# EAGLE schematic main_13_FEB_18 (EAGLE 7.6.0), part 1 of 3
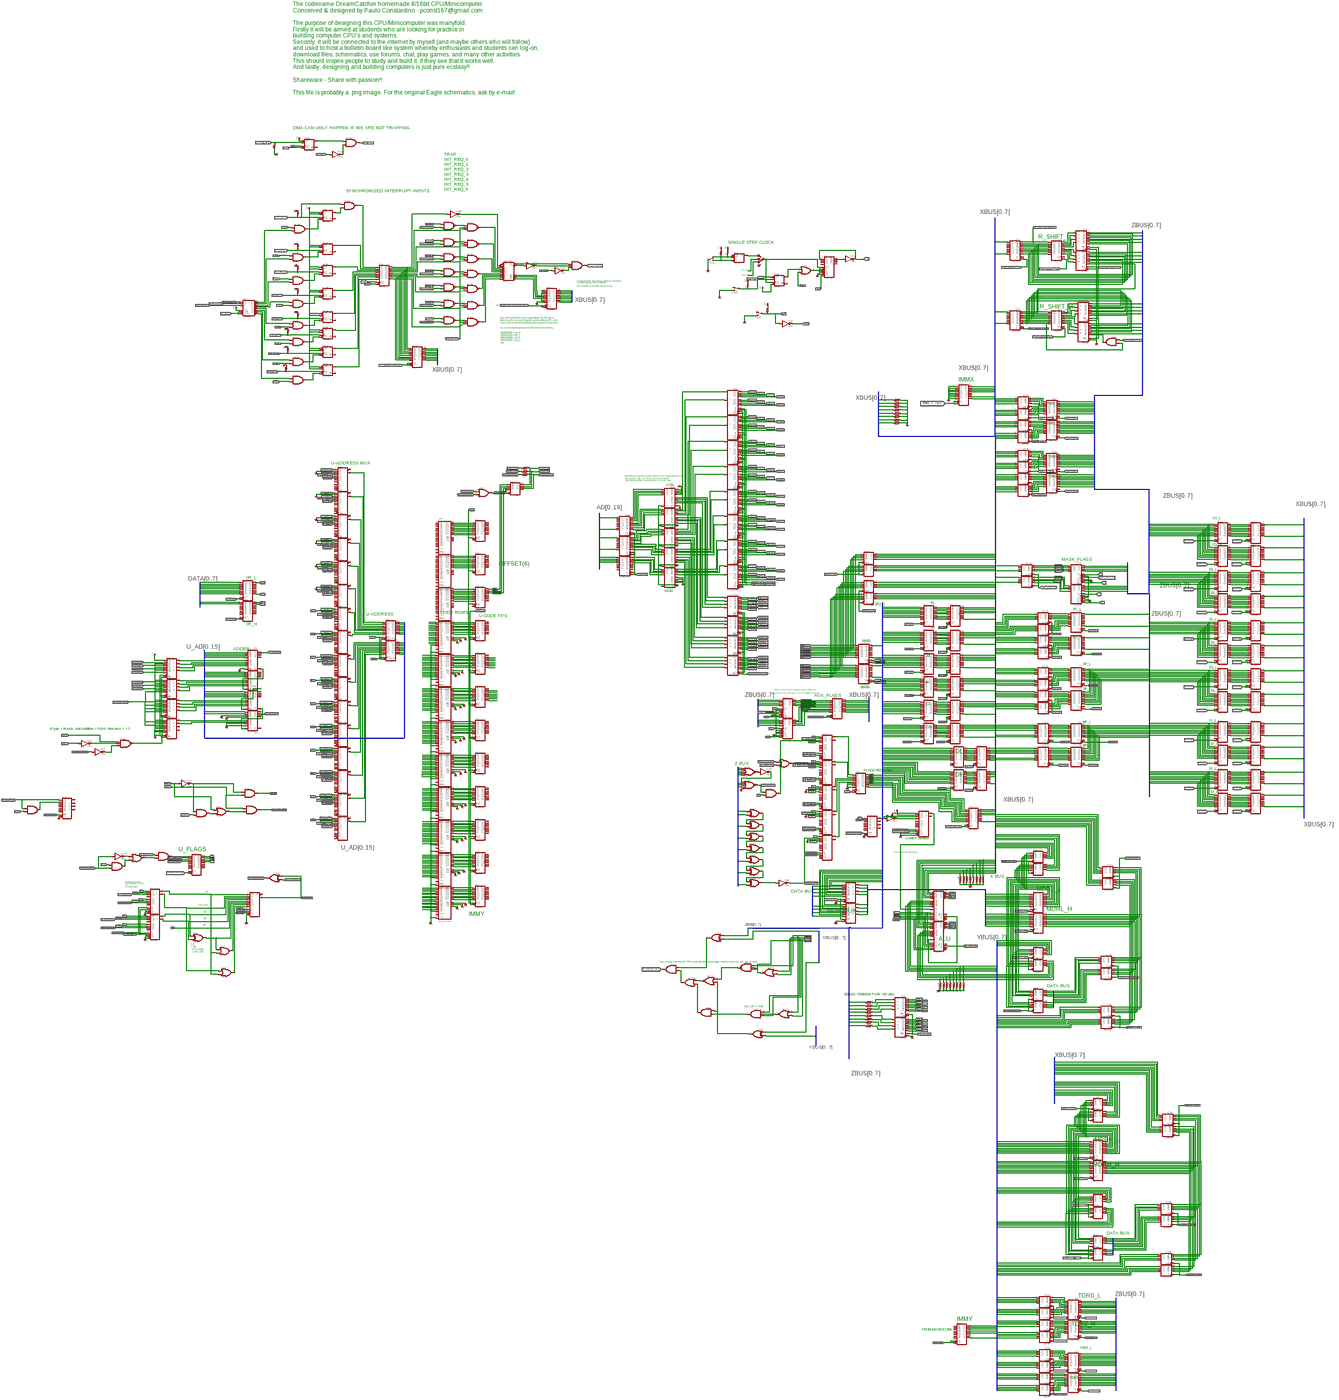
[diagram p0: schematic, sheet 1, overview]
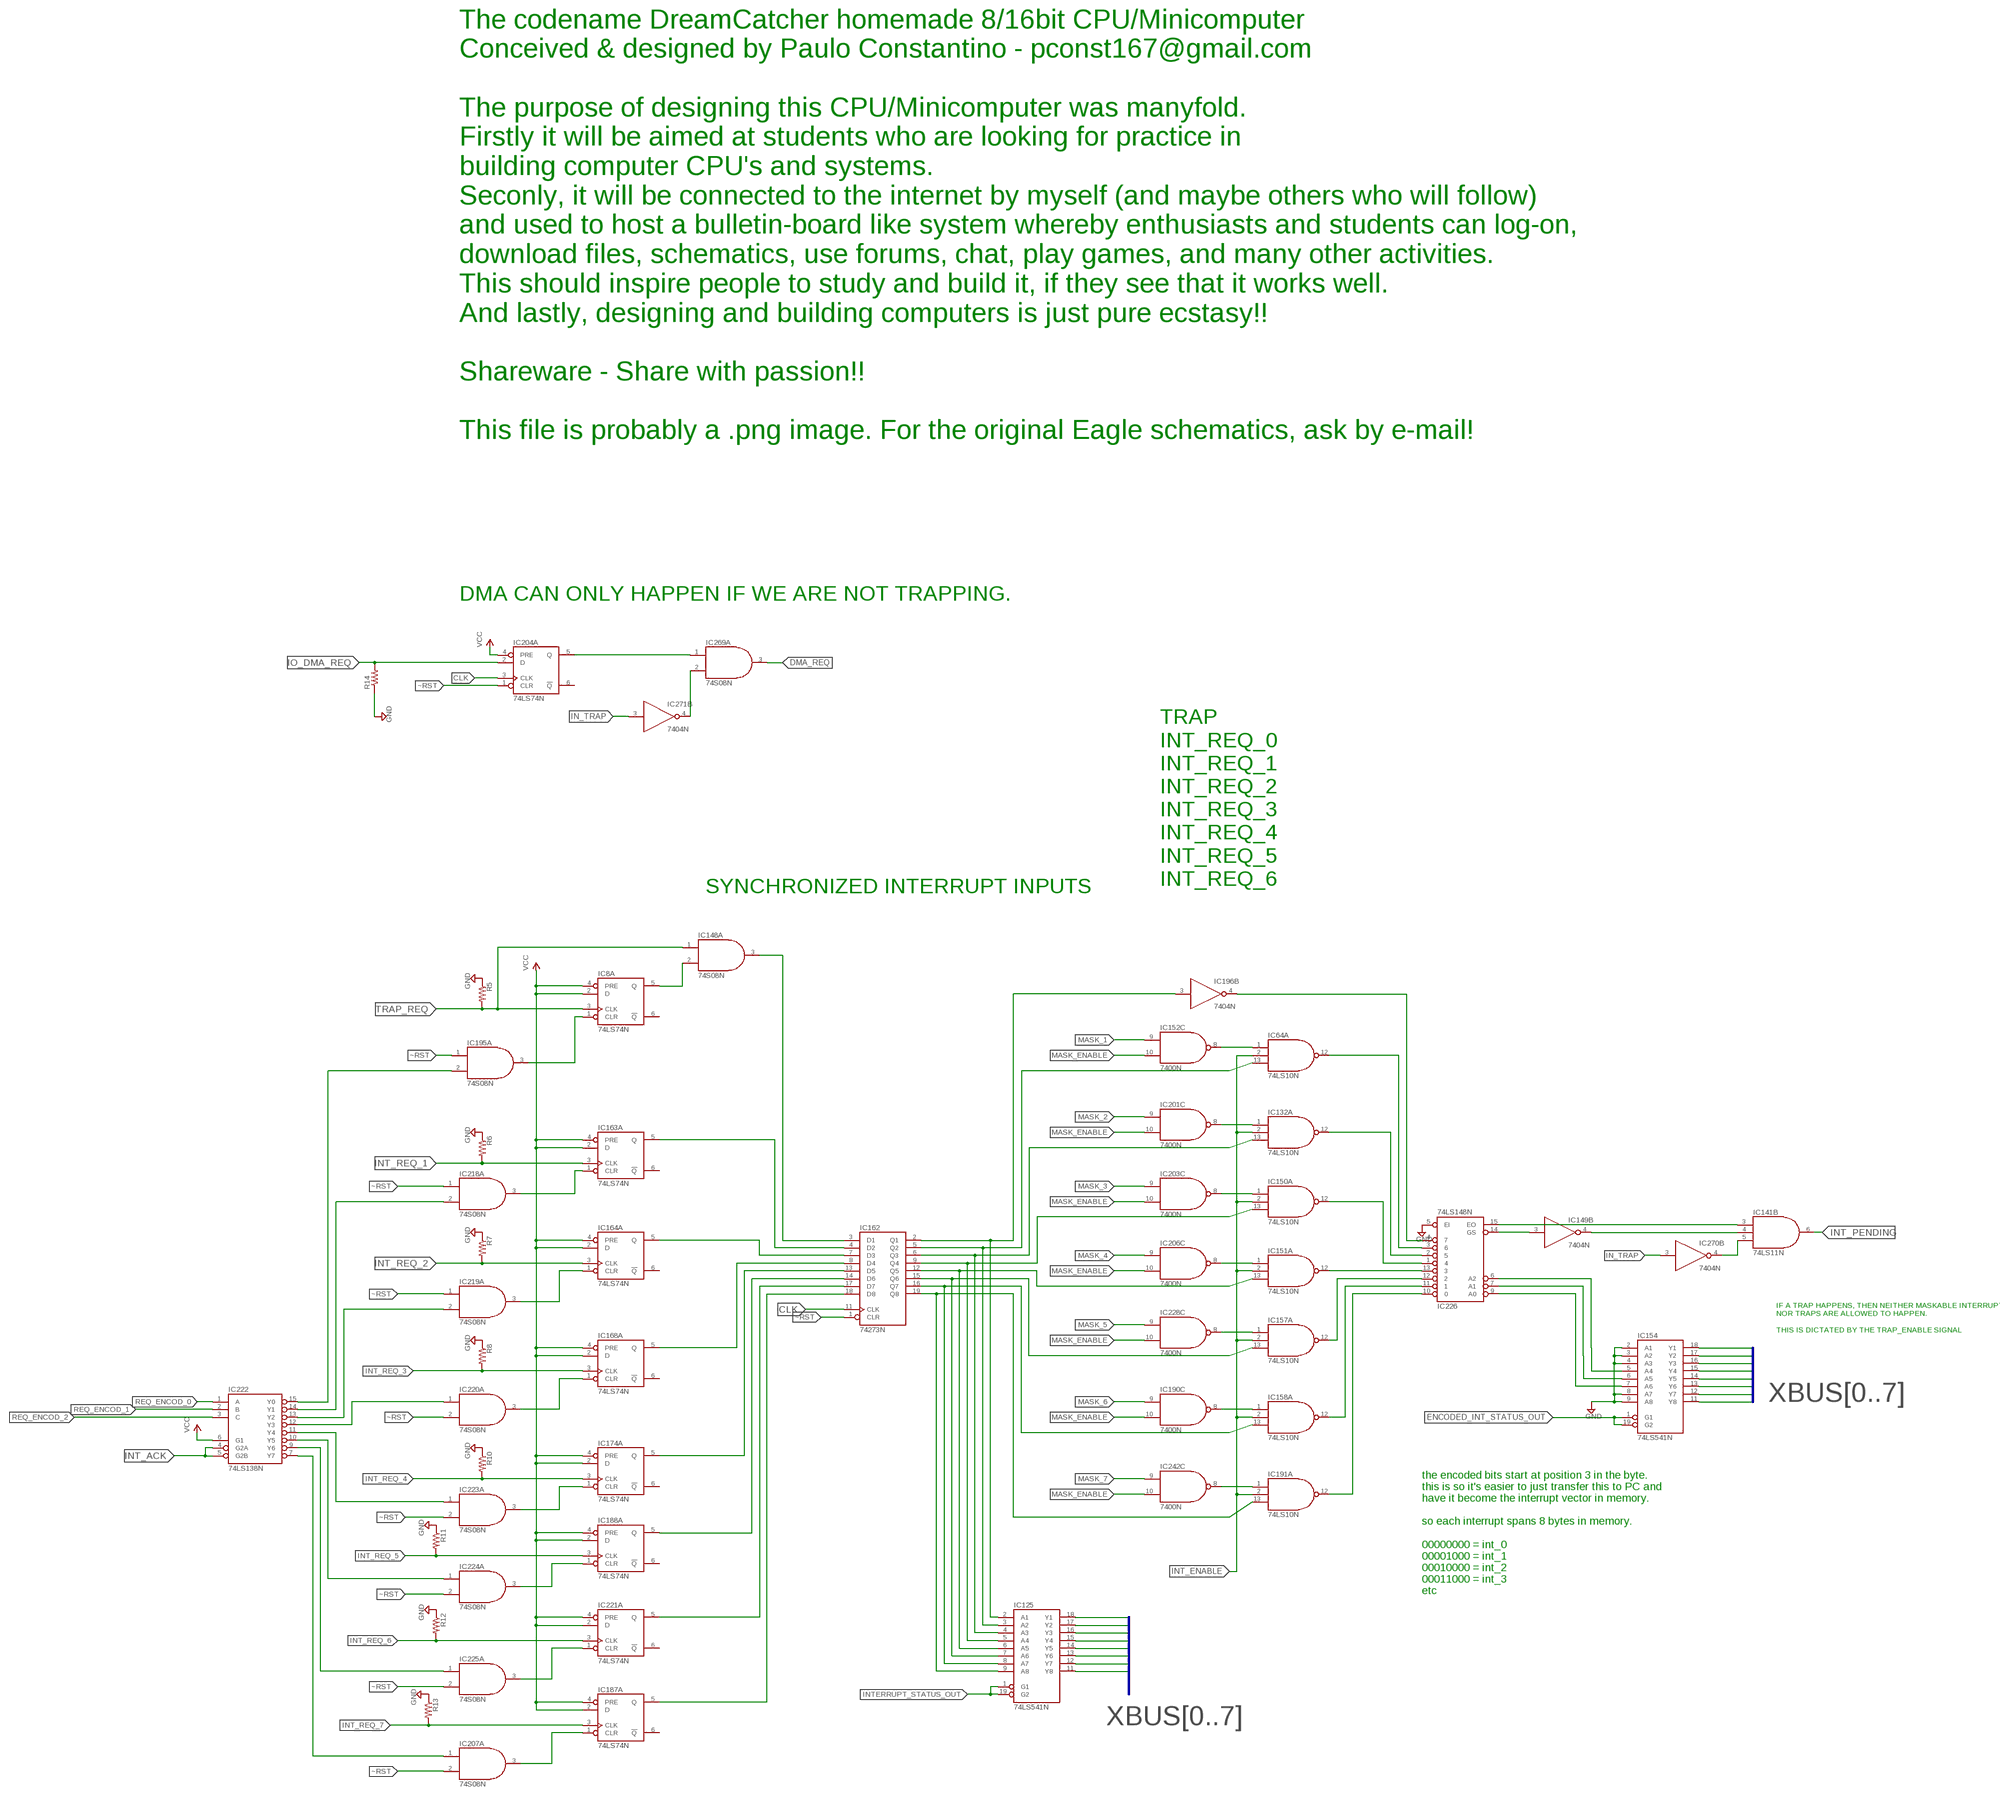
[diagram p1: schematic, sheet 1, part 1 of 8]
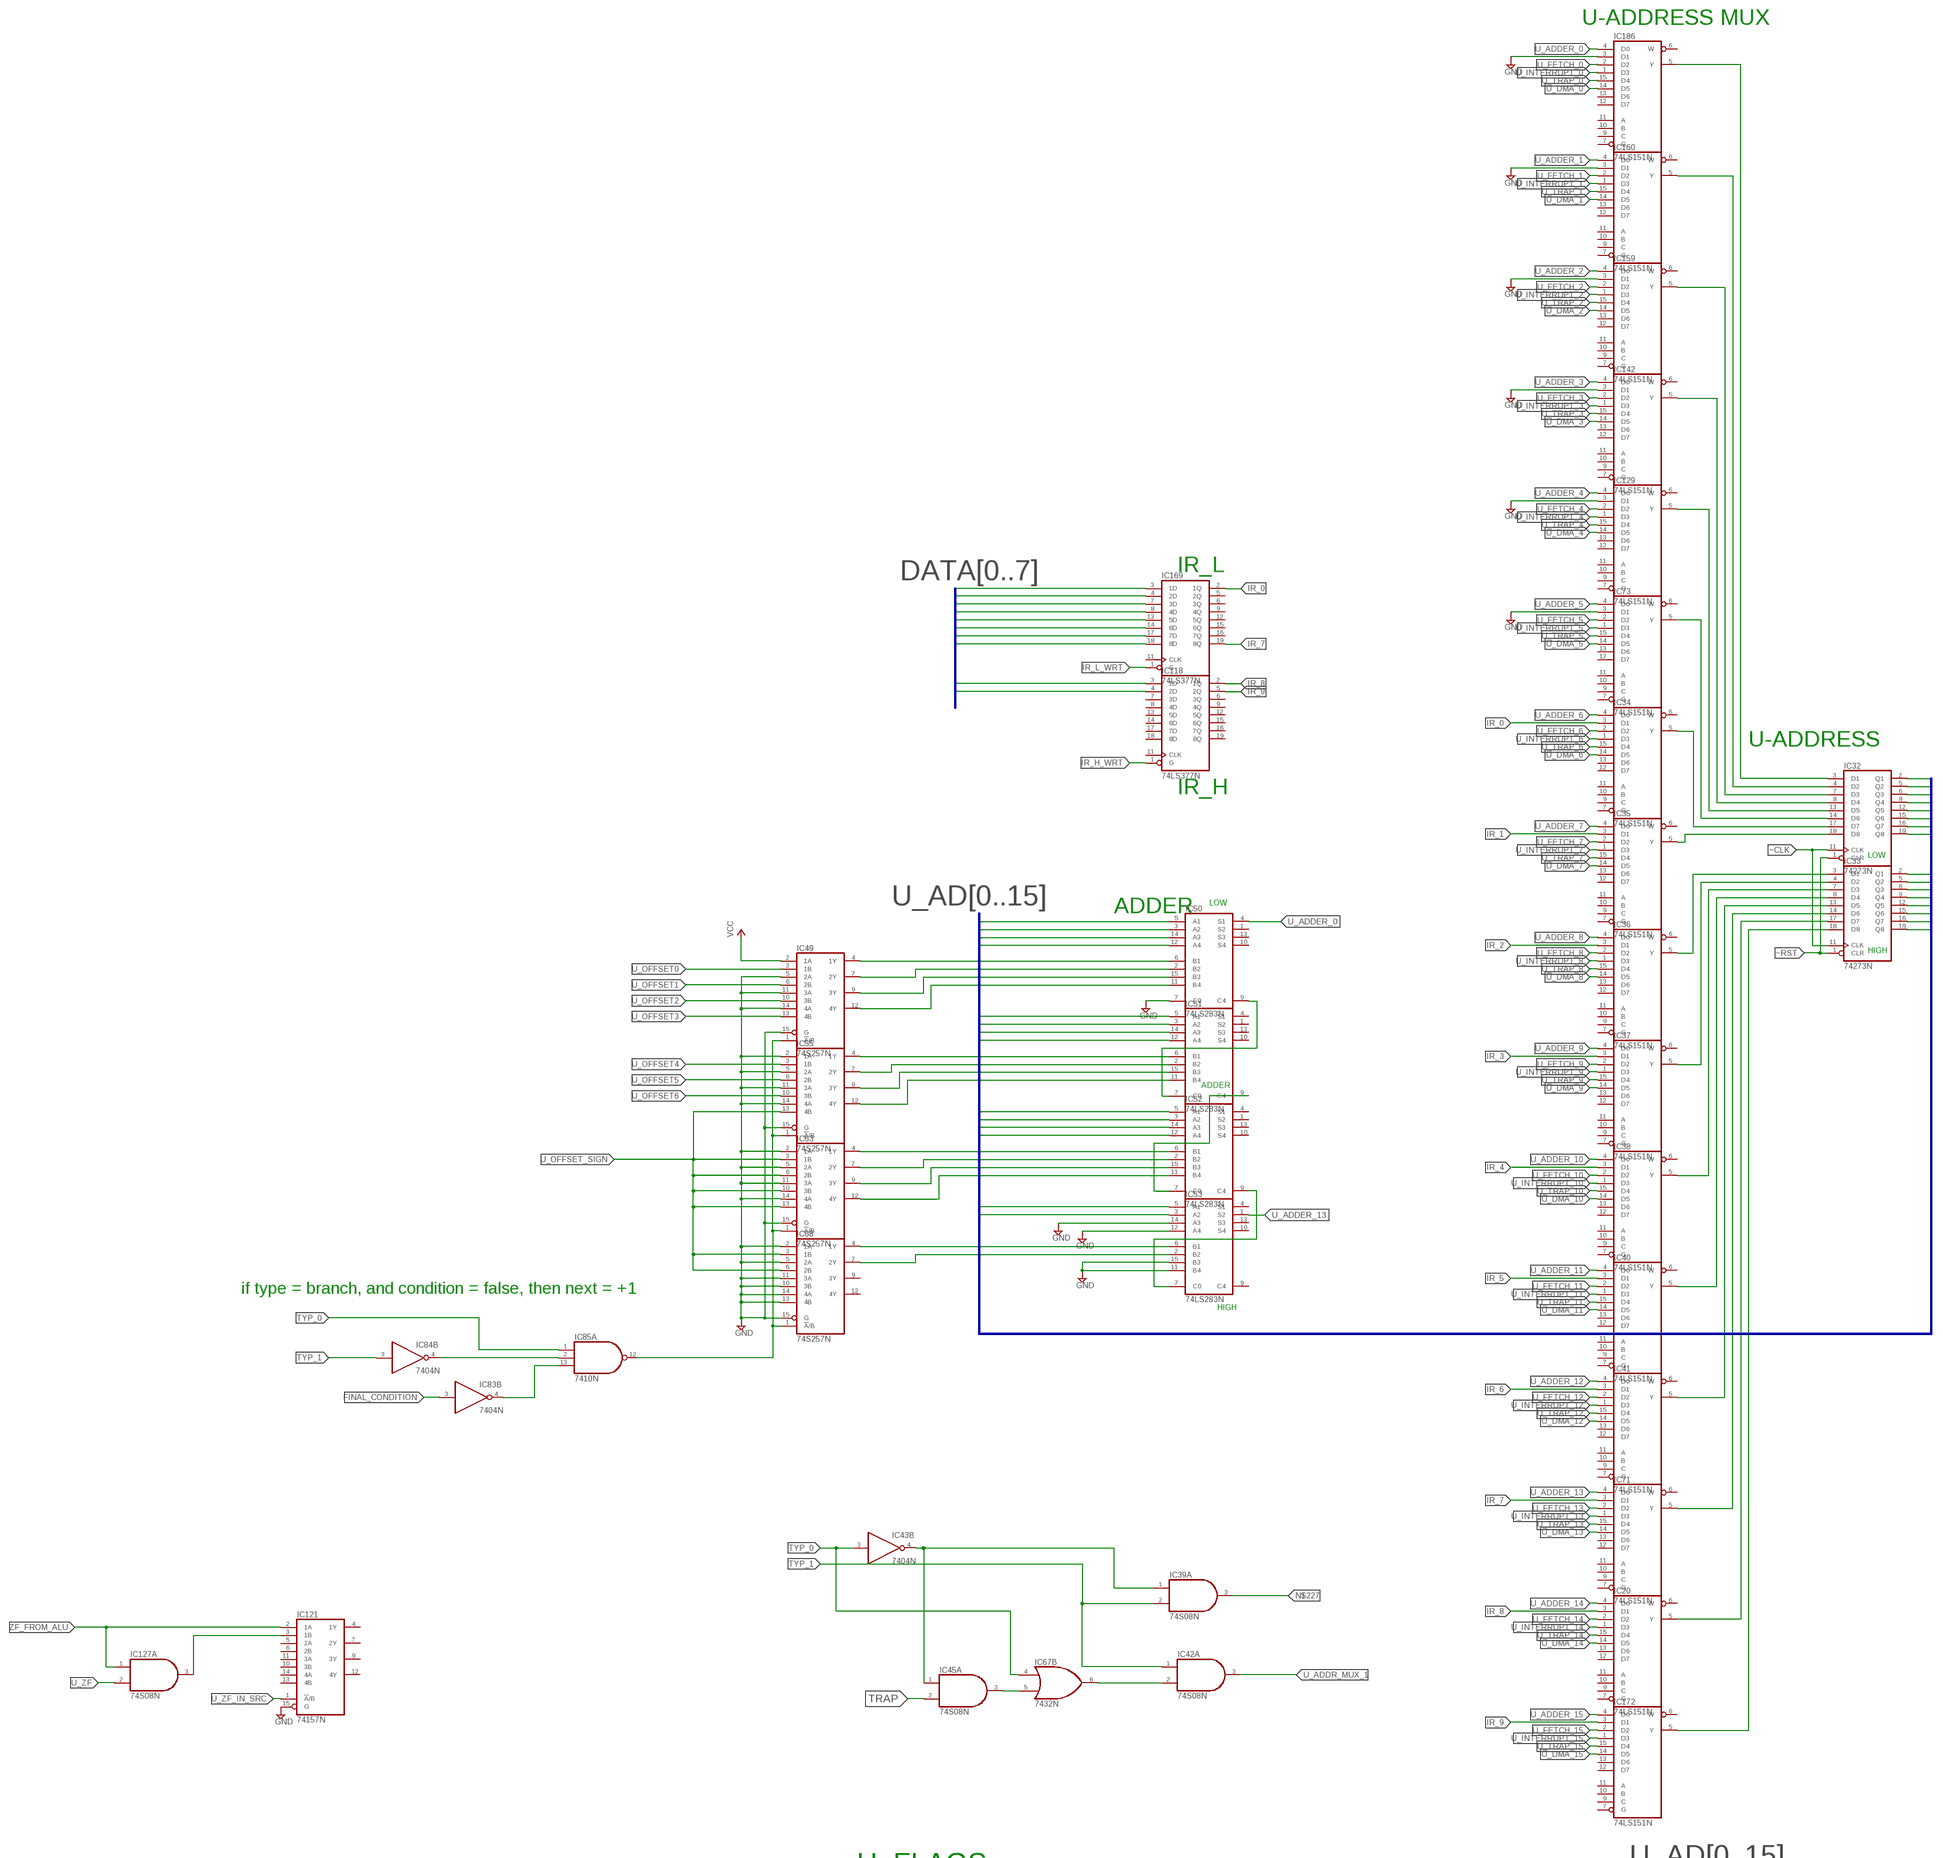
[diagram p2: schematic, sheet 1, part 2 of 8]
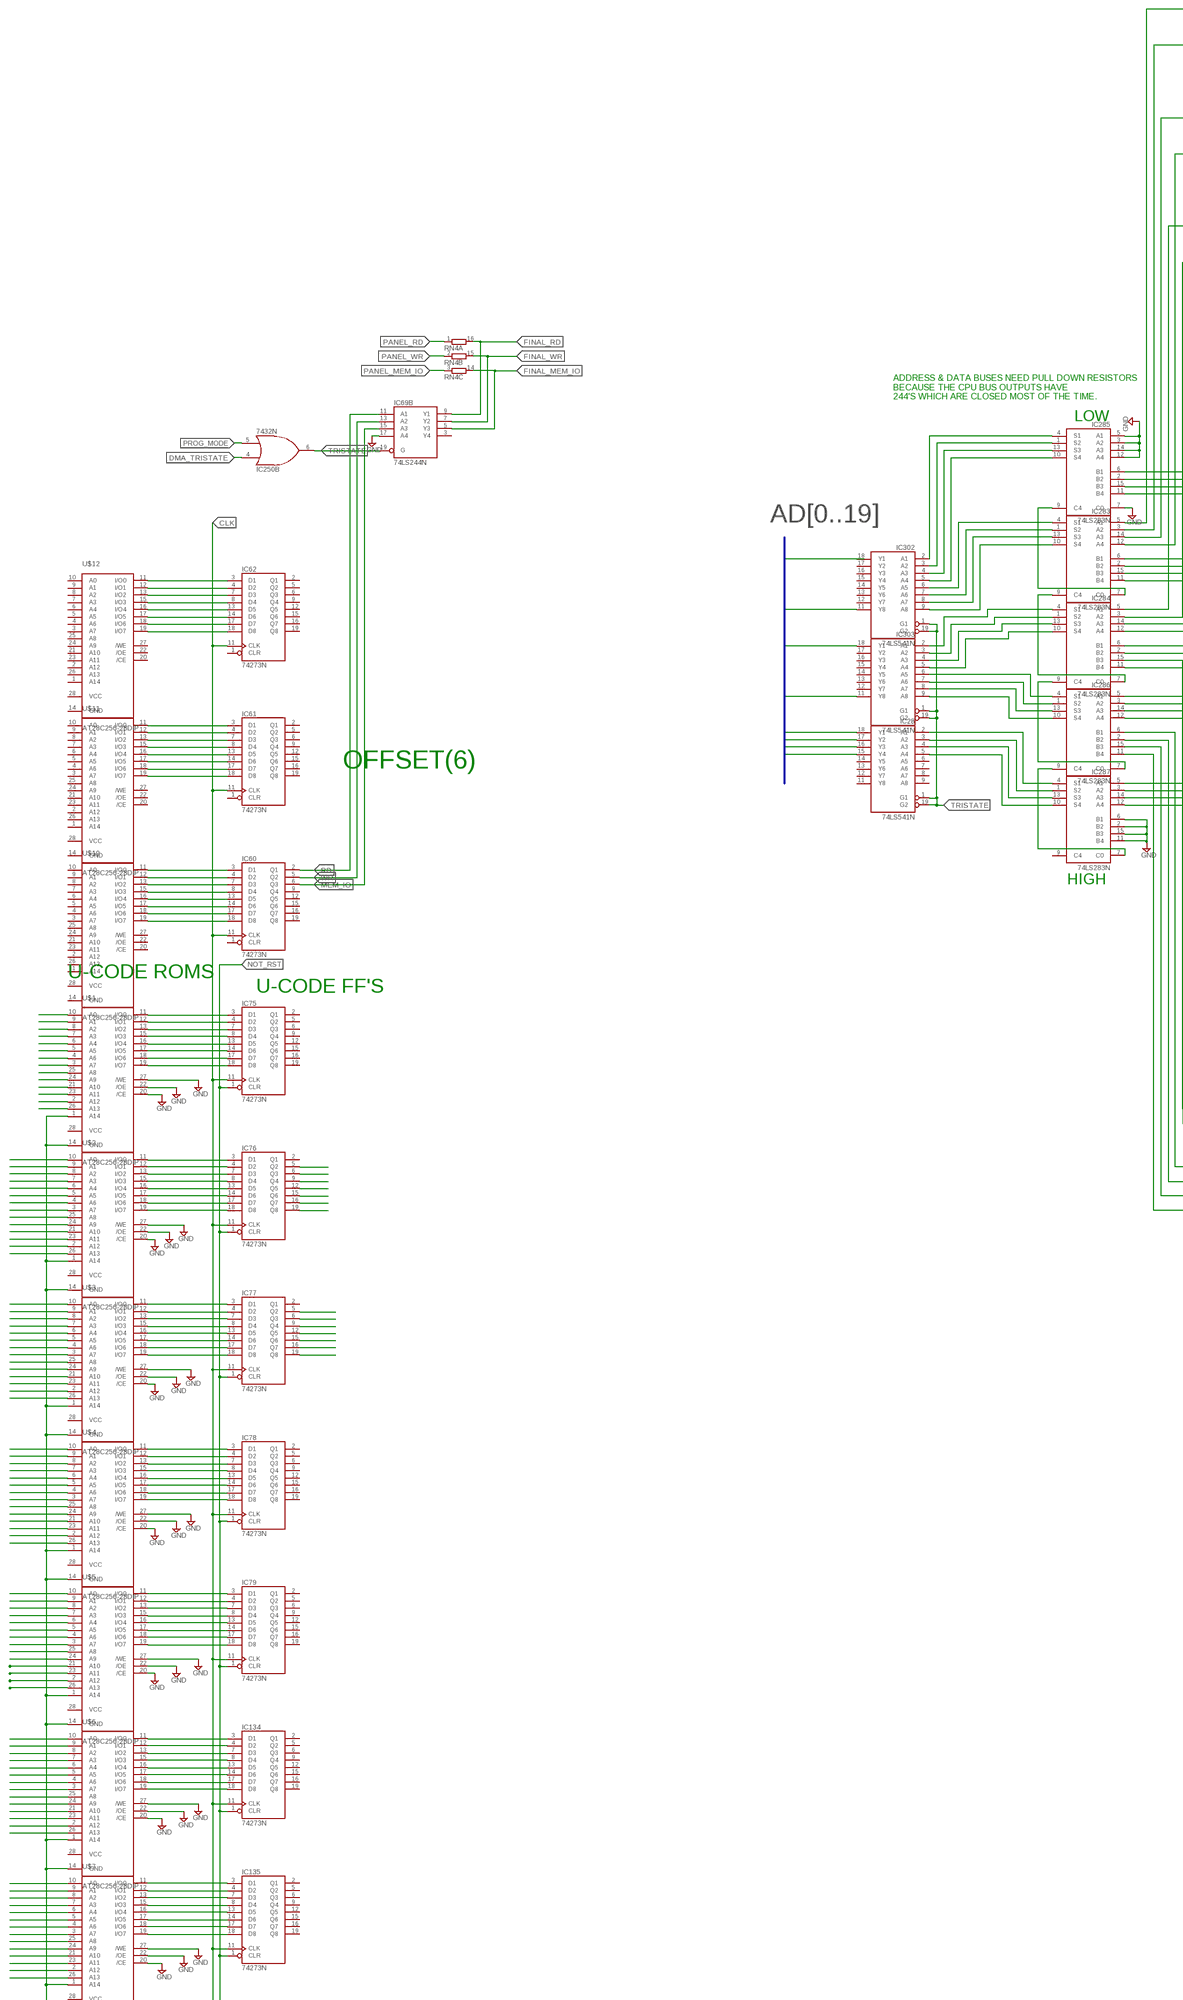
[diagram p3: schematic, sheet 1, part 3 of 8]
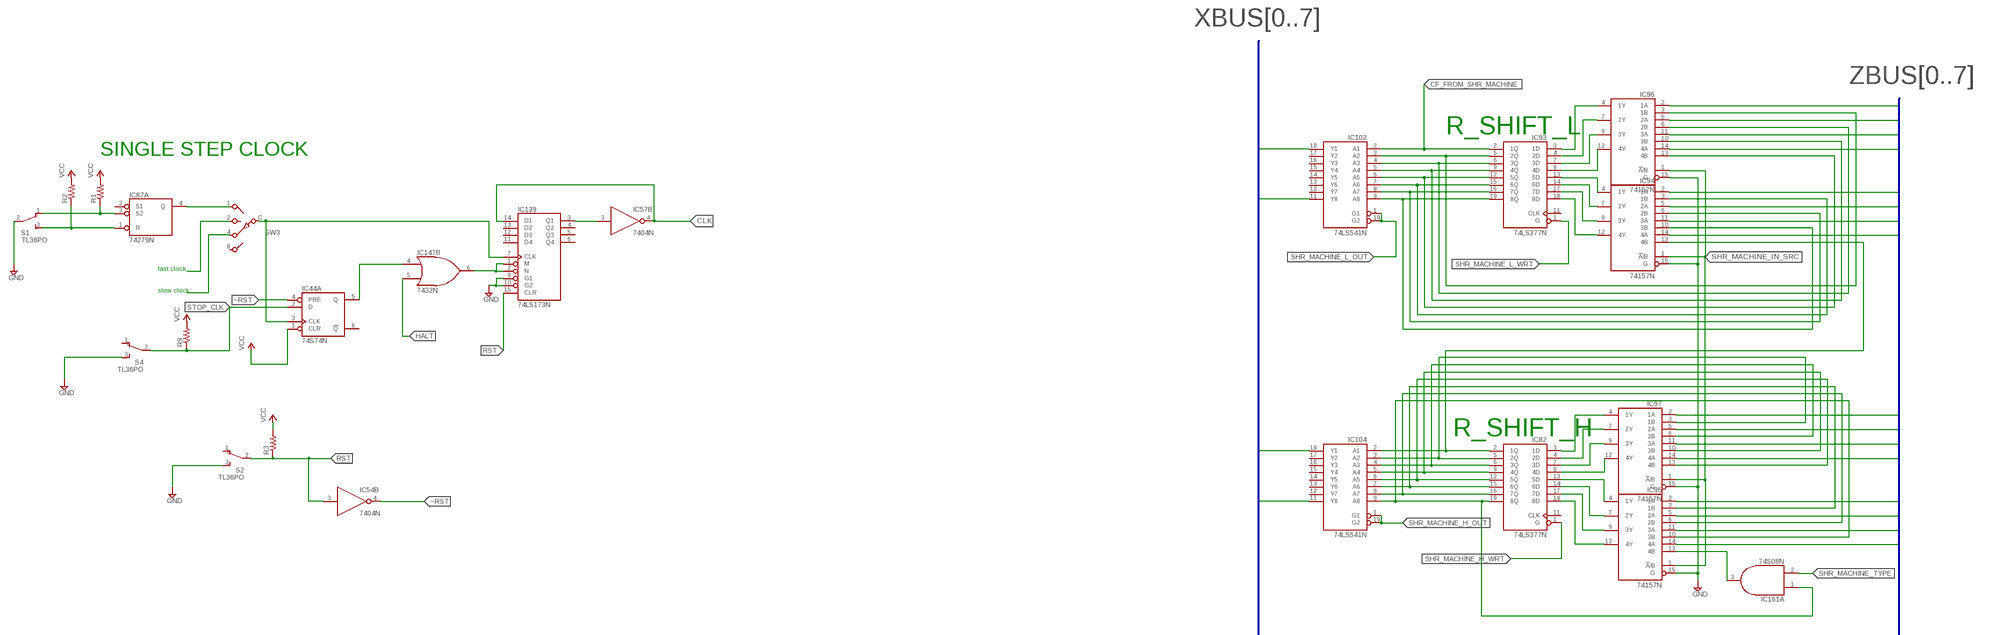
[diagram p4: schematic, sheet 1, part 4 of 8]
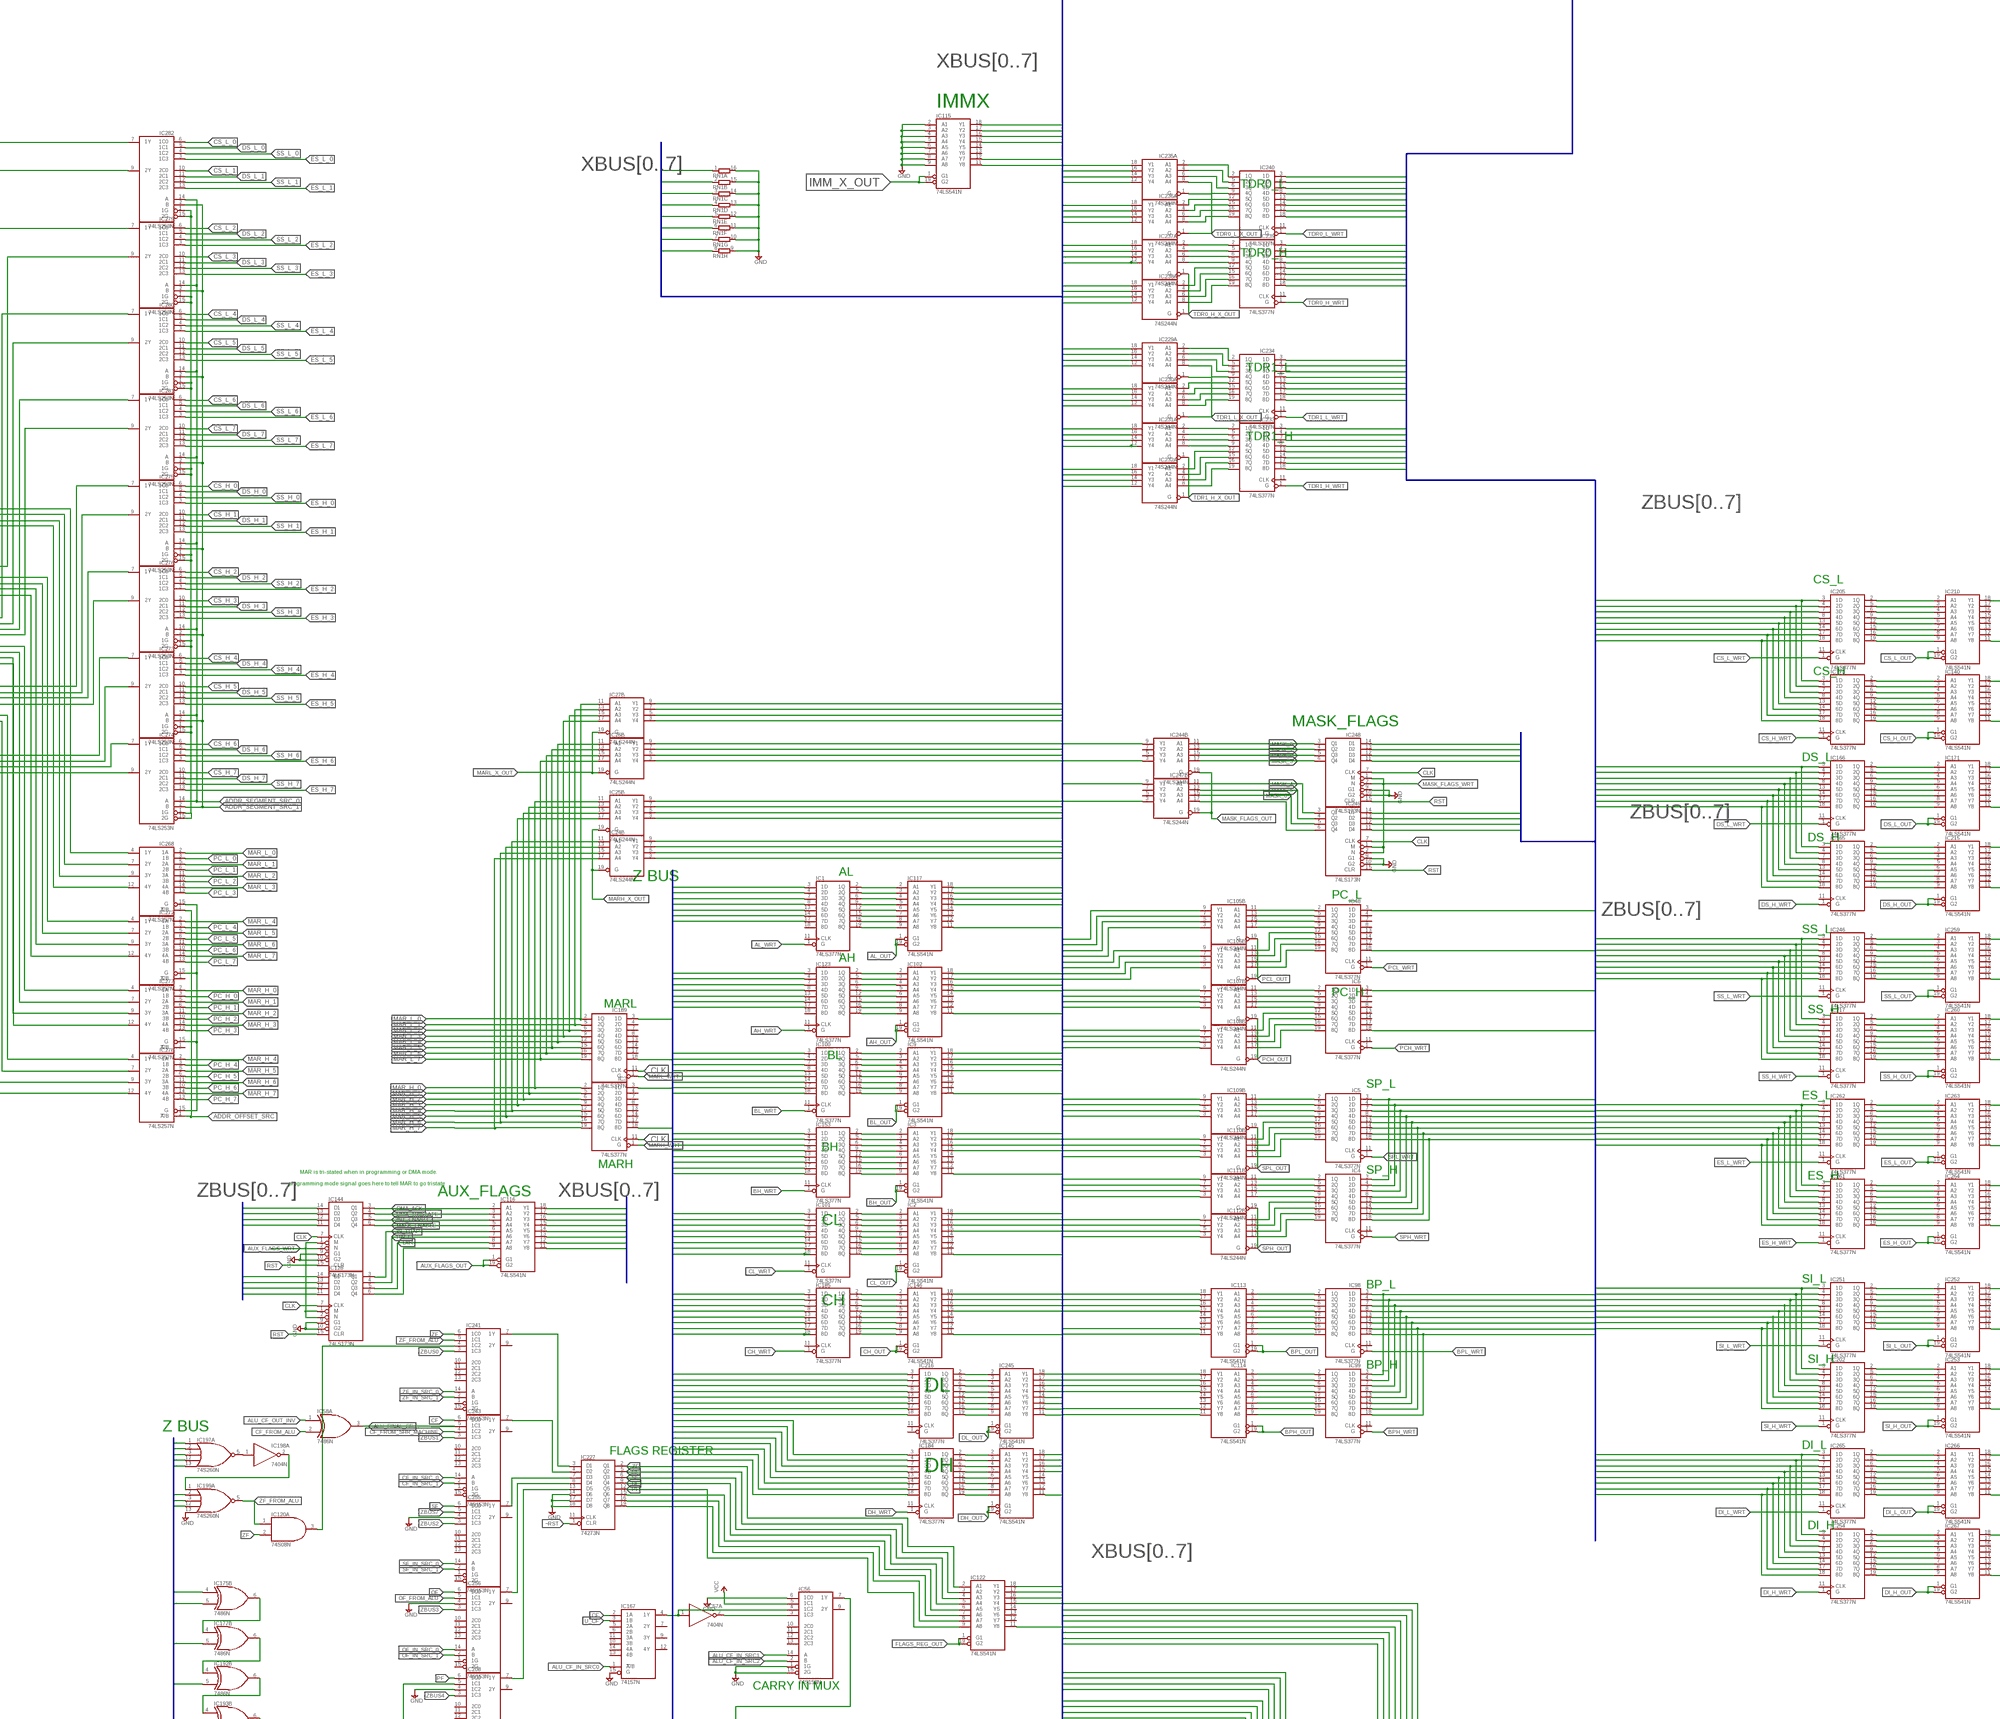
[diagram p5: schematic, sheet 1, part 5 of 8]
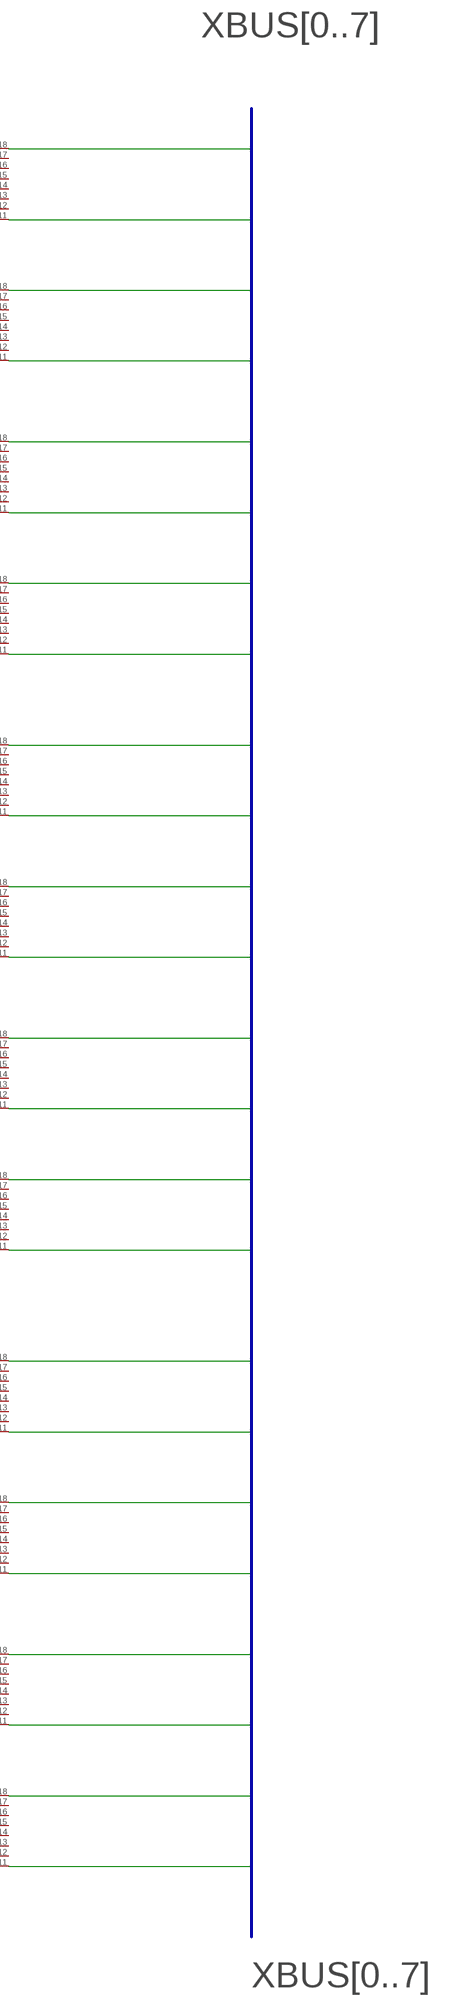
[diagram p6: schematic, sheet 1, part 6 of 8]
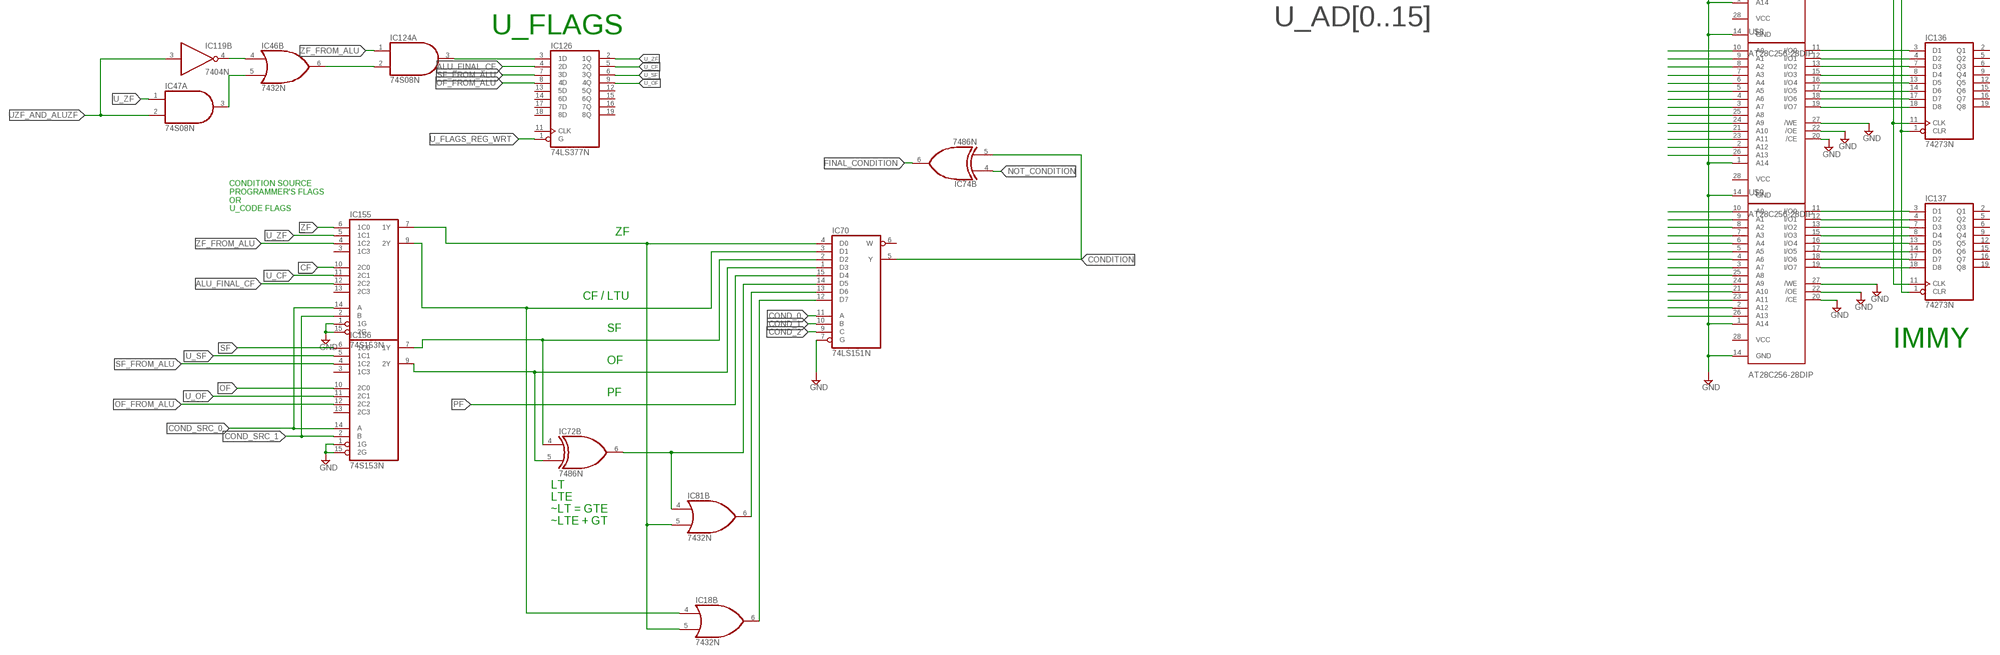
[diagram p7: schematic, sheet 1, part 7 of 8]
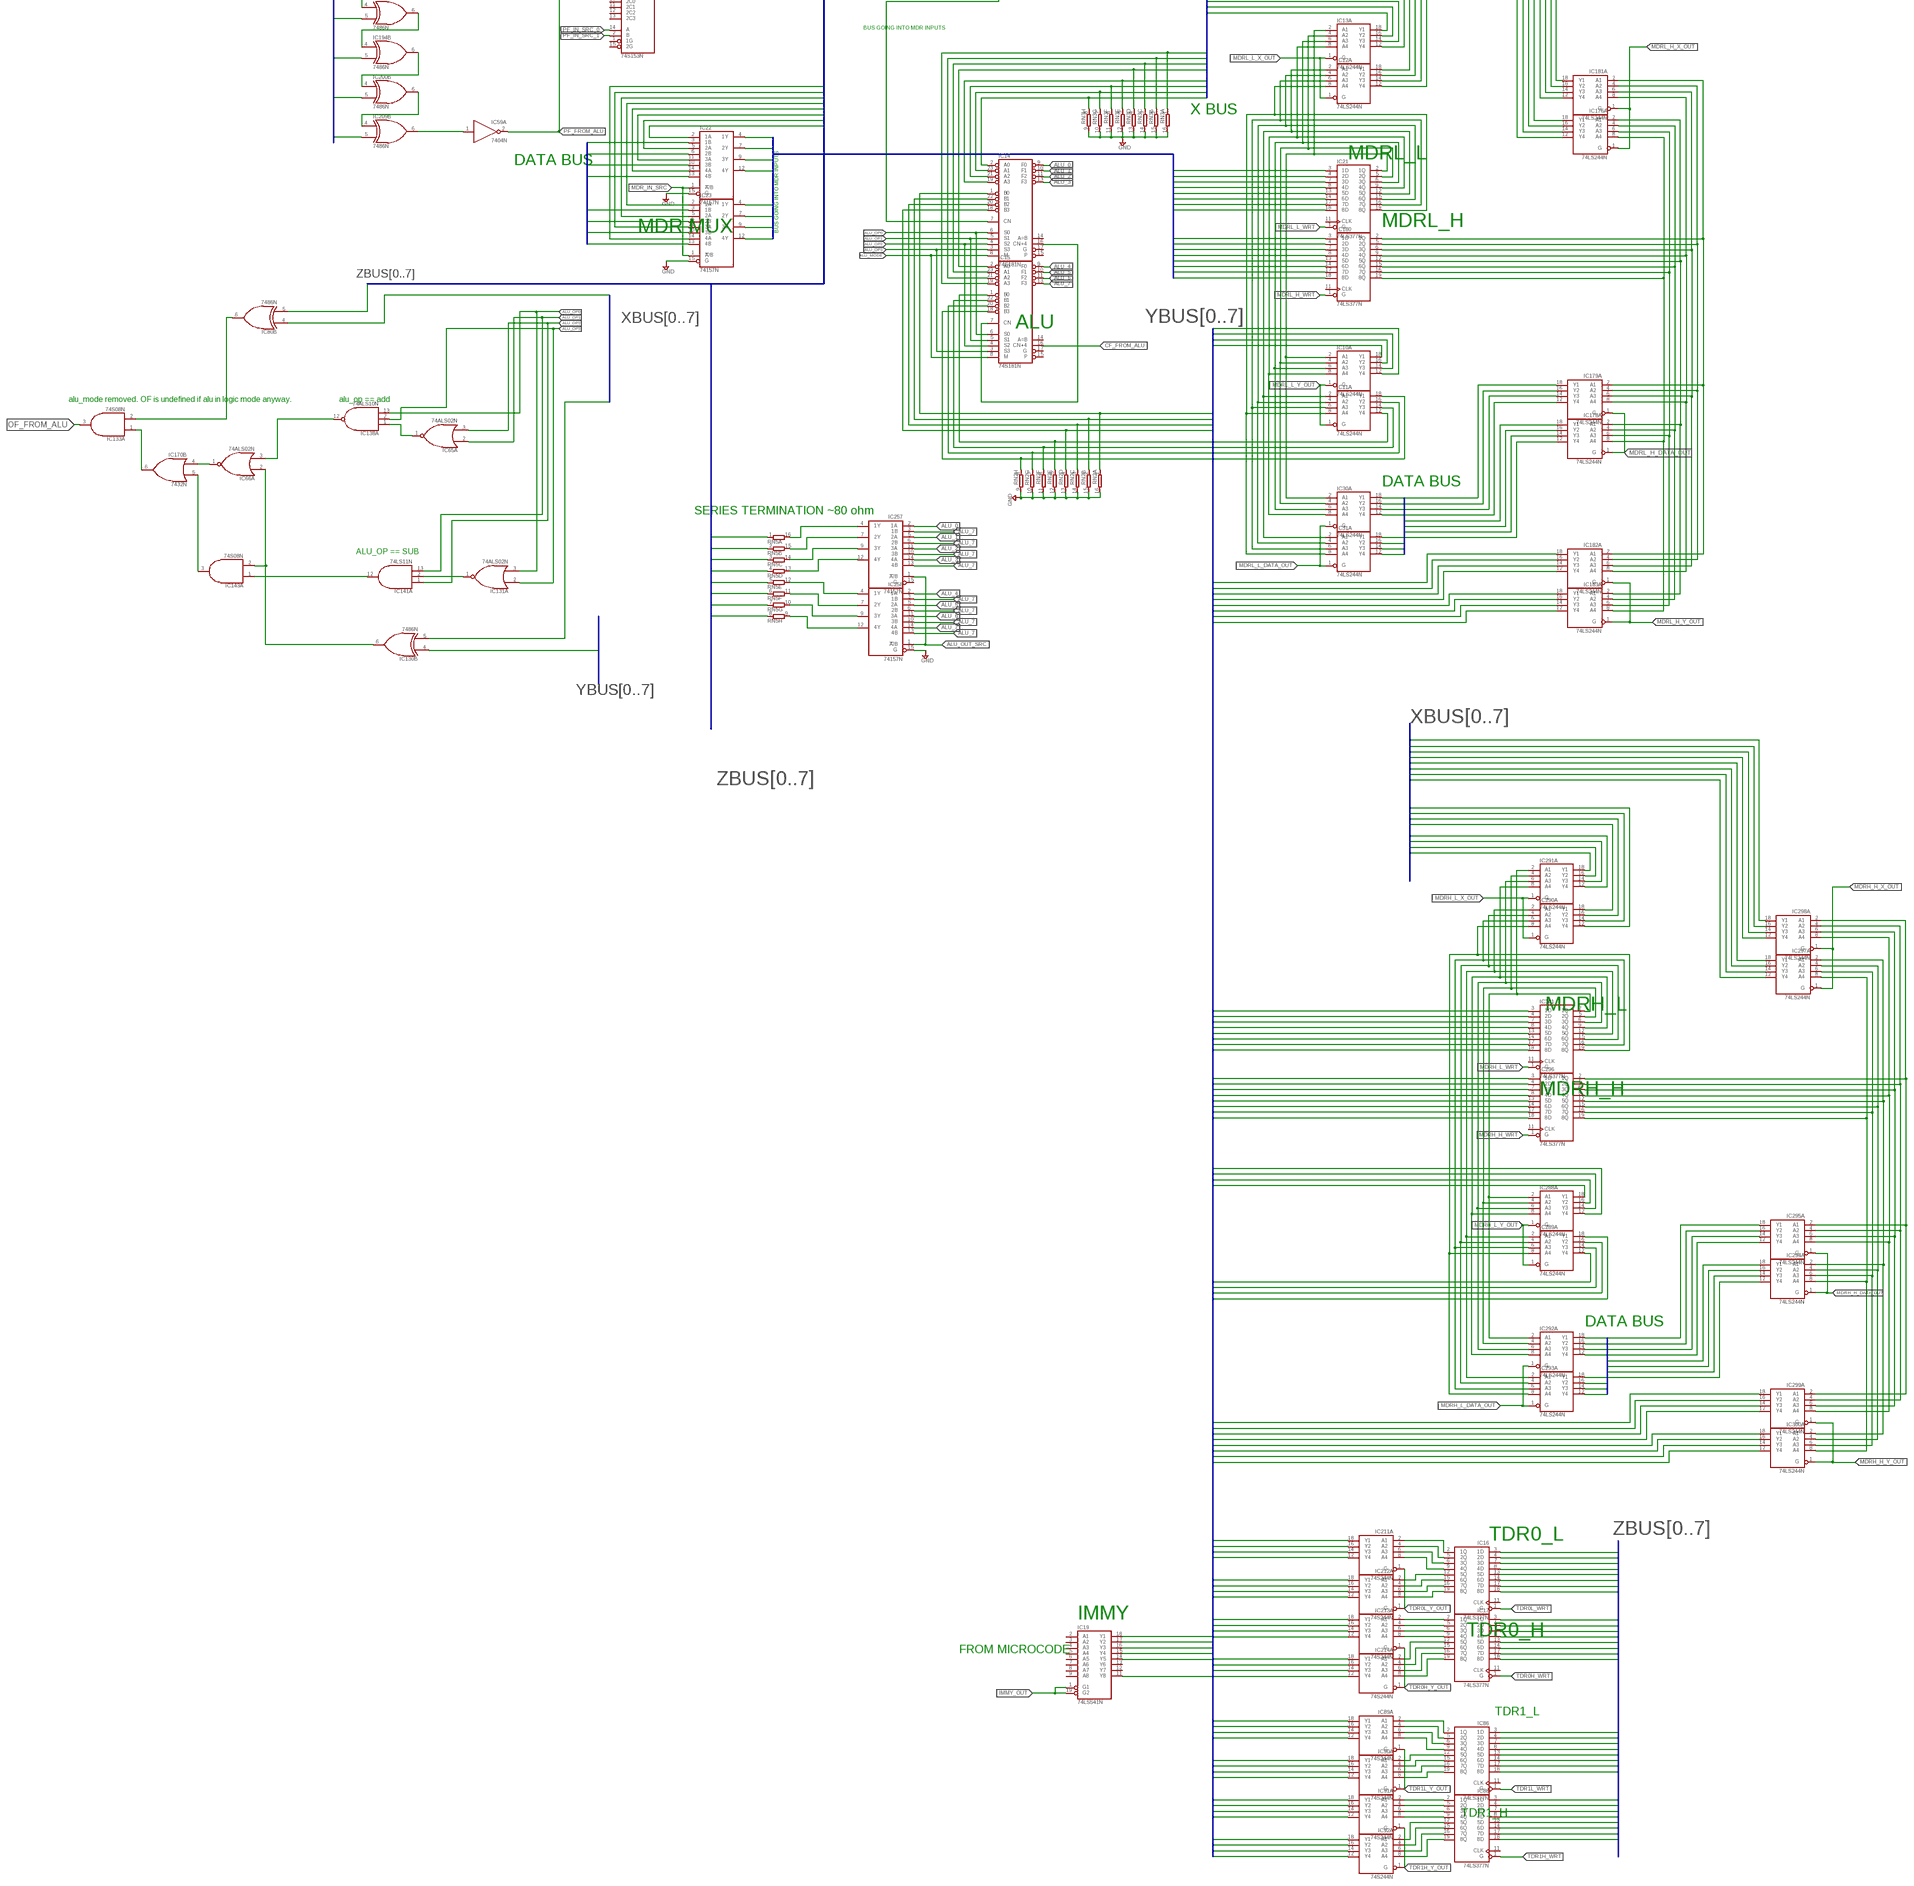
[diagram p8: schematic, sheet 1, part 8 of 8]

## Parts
IC1  74LS377N  [DIL20]
IC2  74LS541N  [DIL20]
IC3  74LS541N  [DIL20]
IC4  74LS377N  [DIL20]
IC5  74LS377N  [DIL20]
IC6  74LS377N  [DIL20]
IC7  74LS377N  [DIL20]
IC8  74LS74N  [DIL14]
IC9  74LS541N  [DIL20]
IC10  74LS244N  [DIL20]
IC11  74LS244N  [DIL20]
IC12  74LS244N  [DIL20]
IC13  74LS244N  [DIL20]
IC14  74S181N  [DIL24-6]
IC15  74S181N  [DIL24-6]
IC16  74LS377N  [DIL20]
IC17  74LS377N  [DIL20]
IC18  7432N  [DIL14]
IC19  74LS541N  [DIL20]
IC20  74LS151N  [DIL16]
IC21  74LS377N  [DIL20]
IC22  74157N  [DIL16]
IC23  74157N  [DIL16]
IC24  74LS244N  [DIL20]
IC25  74LS244N  [DIL20]
IC26  74LS244N  [DIL20]
IC27  74LS244N  [DIL20]
IC28  74LS541N  [DIL20]
IC30  74LS244N  [DIL20]
IC31  74LS244N  [DIL20]
IC32  74273N  [DIL20]
IC33  74273N  [DIL20]
IC34  74LS151N  [DIL16]
IC35  74LS151N  [DIL16]
IC36  74LS151N  [DIL16]
IC37  74LS151N  [DIL16]
IC38  74LS151N  [DIL16]
IC39  74S08N  [DIL14]
IC40  74LS151N  [DIL16]
IC41  74LS151N  [DIL16]
IC42  74S08N  [DIL14]
IC43  7404N  [DIL14]
IC44  74S74N  [DIL14]
IC45  74S08N  [DIL14]
IC46  7432N  [DIL14]
IC47  74S08N  [DIL14]
IC48  74LS377N  [DIL20]
IC49  74S257N  [DIL16]
IC50  74LS283N  [DIL16]
IC51  74LS283N  [DIL16]
IC52  74LS283N  [DIL16]
IC53  74LS283N  [DIL16]
IC54  7404N  [DIL14]
IC55  74S257N  [DIL16]
IC56  74S153N  [DIL16]
IC57  7404N  [DIL14]
IC58  7486N  [DIL14]
IC59  7404N  [DIL14]
IC60  74273N  [DIL20]
IC61  74273N  [DIL20]
IC62  74273N  [DIL20]
IC63  74S257N  [DIL16]
IC64  74LS10N  [DIL14]
IC65  74ALS02N  [DIL14]
IC66  74ALS02N  [DIL14]
IC67  7432N  [DIL14]
IC68  74S257N  [DIL16]
IC69  74LS244N  [DIL20]
IC70  74LS151N  [DIL16]
IC71  74LS151N  [DIL16]
IC72  7486N  [DIL14]
IC73  74LS151N  [DIL16]
IC74  7486N  [DIL14]
IC75  74273N  [DIL20]
IC76  74273N  [DIL20]
IC77  74273N  [DIL20]
IC78  74273N  [DIL20]
IC79  74273N  [DIL20]
IC80  7486N  [DIL14]
IC81  7432N  [DIL14]
IC82  74LS377N  [DIL20]
IC83  7404N  [DIL14]
IC84  7404N  [DIL14]
IC85  7410N  [DIL14]
IC86  74LS377N  [DIL20]
IC87  74279N  [DIL16]
IC88  74LS377N  [DIL20]
IC89  74S244N  [DIL20]
IC90  74S244N  [DIL20]
IC91  74S244N  [DIL20]
IC92  74S244N  [DIL20]
IC93  74LS377N  [DIL20]
IC94  74157N  [DIL16]
IC95  74157N  [DIL16]
IC96  74157N  [DIL16]
IC97  74157N  [DIL16]
IC98  74LS377N  [DIL20]
IC99  74LS377N  [DIL20]
IC100  74LS377N  [DIL20]
IC101  74LS377N  [DIL20]
IC102  74LS541N  [DIL20]
IC103  74LS541N  [DIL20]
IC104  74LS541N  [DIL20]
IC105  74LS244N  [DIL20]
IC106  74LS244N  [DIL20]
IC107  74LS244N  [DIL20]
IC108  74LS244N  [DIL20]
IC109  74LS244N  [DIL20]
IC110  74LS244N  [DIL20]
IC111  74LS244N  [DIL20]
IC112  74LS244N  [DIL20]
IC113  74LS541N  [DIL20]
IC114  74LS541N  [DIL20]
IC115  74LS541N  [DIL20]
IC116  74LS541N  [DIL20]
IC117  74LS541N  [DIL20]
IC118  74LS377N  [DIL20]
IC119  7404N  [DIL14]
IC120  74S08N  [DIL14]
IC121  74157N  [DIL16]
IC122  74LS541N  [DIL20]
IC123  74LS377N  [DIL20]
IC124  74S08N  [DIL14]
IC125  74LS541N  [DIL20]
IC126  74LS377N  [DIL20]
IC127  74S08N  [DIL14]
IC128  74LS173N  [DIL16]
IC129  74LS151N  [DIL16]
IC130  7486N  [DIL14]
IC131  74ALS02N  [DIL14]
IC132  74LS10N  [DIL14]
IC133  74S08N  [DIL14]
IC134  74273N  [DIL20]
IC135  74273N  [DIL20]
IC136  74273N  [DIL20]
IC137  74273N  [DIL20]
IC138  74ALS10N  [DIL14]
IC139  74LS173N  [DIL16]
IC140  74LS541N  [DIL20]
IC141  74LS11N  [DIL14]
IC142  74LS151N  [DIL16]
IC143  74S08N  [DIL14]
IC144  74LS173N  [DIL16]
IC145  74LS541N  [DIL20]
IC146  74LS541N  [DIL20]
IC147  7432N  [DIL14]
IC148  74S08N  [DIL14]
IC149  7404N  [DIL14]
IC150  74LS10N  [DIL14]
IC151  74LS10N  [DIL14]
IC152  7400N  [DIL14]
IC153  74LS377N  [DIL20]
IC154  74LS541N  [DIL20]
IC155  74S153N  [DIL16]
IC156  74S153N  [DIL16]
IC157  74LS10N  [DIL14]
IC158  74LS10N  [DIL14]
IC159  74LS151N  [DIL16]
IC160  74LS151N  [DIL16]
IC161  74S08N  [DIL14]
IC162  74273N  [DIL20]
IC163  74LS74N  [DIL14]
IC164  74LS74N  [DIL14]
IC165  74LS377N  [DIL20]
IC166  74LS377N  [DIL20]
IC167  74157N  [DIL16]
IC168  74LS74N  [DIL14]
IC169  74LS377N  [DIL20]
IC170  7432N  [DIL14]
IC171  74LS541N  [DIL20]
IC172  74LS151N  [DIL16]
IC173  74LS377N  [DIL20]
IC174  74LS74N  [DIL14]
IC175  7486N  [DIL14]
IC176  74LS244N  [DIL20]
IC177  7486N  [DIL14]
IC178  74LS244N  [DIL20]
IC179  74LS244N  [DIL20]
IC180  74LS377N  [DIL20]
IC181  74LS244N  [DIL20]
IC182  74LS244N  [DIL20]
IC183  74LS244N  [DIL20]
IC184  74LS377N  [DIL20]
IC185  74LS377N  [DIL20]
IC186  74LS151N  [DIL16]
IC187  74LS74N  [DIL14]
IC188  74LS74N  [DIL14]
IC189  74LS377N  [DIL20]
IC190  7400N  [DIL14]
IC191  74LS10N  [DIL14]
IC192  7486N  [DIL14]
IC193  7486N  [DIL14]
IC194  7486N  [DIL14]
IC195  74S08N  [DIL14]
IC196  7404N  [DIL14]
IC197  74S260N  [DIL14]
IC198  7404N  [DIL14]
IC199  74S260N  [DIL14]
IC200  7486N  [DIL14]
IC201  7400N  [DIL14]
IC202  74LS377N  [DIL20]
IC203  7400N  [DIL14]
IC204  74LS74N  [DIL14]
IC205  74LS377N  [DIL20]
IC206  7400N  [DIL14]
IC207  74S08N  [DIL14]
IC208  74S153N  [DIL16]
IC209  7486N  [DIL14]
IC210  74LS541N  [DIL20]
IC211  74S244N  [DIL20]
IC212  74S244N  [DIL20]
IC213  74S244N  [DIL20]
IC214  74S244N  [DIL20]
IC215  74LS541N  [DIL20]
IC216  74LS377N  [DIL20]
IC217  74LS377N  [DIL20]
IC218  74S08N  [DIL14]
IC219  74S08N  [DIL14]
IC220  74S08N  [DIL14]
IC221  74LS74N  [DIL14]
IC222  74LS138N  [DIL16]
IC223  74S08N  [DIL14]
IC224  74S08N  [DIL14]
IC225  74S08N  [DIL14]
IC226  74LS148N  [DIL16]
IC227  74273N  [DIL20]
IC228  7400N  [DIL14]
IC229  74S244N  [DIL20]
IC230  74S244N  [DIL20]
IC231  74S244N  [DIL20]
IC232  74S244N  [DIL20]
IC233  74LS377N  [DIL20]
IC234  74LS377N  [DIL20]
IC235  74S244N  [DIL20]
IC236  74S244N  [DIL20]
IC237  74S244N  [DIL20]
IC238  74S244N  [DIL20]
IC239  74LS377N  [DIL20]
IC240  74LS377N  [DIL20]
IC241  74S153N  [DIL16]
IC242  7400N  [DIL14]
IC243  74S153N  [DIL16]
IC244  74LS244N  [DIL20]
IC245  74LS541N  [DIL20]
IC246  74LS377N  [DIL20]
IC247  74LS244N  [DIL20]
IC248  74LS173N  [DIL16]
IC249  74LS173N  [DIL16]
IC250  7432N  [DIL14]
IC251  74LS377N  [DIL20]
IC252  74LS541N  [DIL20]
IC253  74LS541N  [DIL20]
IC254  74LS377N  [DIL20]
IC255  74S153N  [DIL16]
IC256  74S153N  [DIL16]
IC257  74157N  [DIL16]
IC258  74157N  [DIL16]
IC259  74LS541N  [DIL20]
IC260  74LS541N  [DIL20]
IC261  74LS377N  [DIL20]
IC262  74LS377N  [DIL20]
IC263  74LS541N  [DIL20]
IC264  74LS541N  [DIL20]
IC265  74LS377N  [DIL20]
IC266  74LS541N  [DIL20]
IC267  74LS541N  [DIL20]
IC268  74LS257N  [DIL16]
IC269  74S08N  [DIL14]
IC270  7404N  [DIL14]
IC271  7404N  [DIL14]
IC272  74LS257N  [DIL16]
IC273  74LS253N  [DIL16]
IC274  74LS253N  [DIL16]
IC275  74LS253N  [DIL16]
IC276  74LS253N  [DIL16]
IC277  74LS257N  [DIL16]
IC278  74LS257N  [DIL16]
IC279  74LS253N  [DIL16]
IC280  74LS253N  [DIL16]
IC281  74LS253N  [DIL16]
IC282  74LS253N  [DIL16]
IC283  74LS283N  [DIL16]
IC284  74LS283N  [DIL16]
IC285  74LS283N  [DIL16]
IC286  74LS283N  [DIL16]
IC287  74LS283N  [DIL16]
IC288  74LS244N  [DIL20]
IC289  74LS244N  [DIL20]
IC290  74LS244N  [DIL20]
IC291  74LS244N  [DIL20]
IC292  74LS244N  [DIL20]
IC293  74LS244N  [DIL20]
IC294  74LS244N  [DIL20]
IC295  74LS244N  [DIL20]
IC296  74LS377N  [DIL20]
IC297  74LS244N  [DIL20]
IC298  74LS244N  [DIL20]
IC299  74LS244N  [DIL20]
IC300  74LS244N  [DIL20]
IC301  74LS377N  [DIL20]
IC302  74LS541N  [DIL20]
IC303  74LS541N  [DIL20]
R1  R-US_0204/2V  [0204V]
R2  R-US_0204/2V  [0204V]
R3  R-US_0204/2V  [0204V]
R5  R-US_0204/7  [0204/7]
R6  R-US_0204/7  [0204/7]
R7  R-US_0204/7  [0204/7]
R8  R-US_0204/7  [0204/7]
R9  R-US_0204/2V  [0204V]
R10  R-US_0204/7  [0204/7]
R11  R-US_0204/7  [0204/7]
R12  R-US_0204/7  [0204/7]
R13  R-US_0204/7  [0204/7]
R14  R-US_0204/7  [0204/7]
RN1  8R-N  [DIL16]
RN2  8R-N  [DIL16]
RN3  8R-N  [DIL16]
RN4  8R-N  [DIL16]
RN5  8R-N  [DIL16]
S1  TL36PO  [TL3XPO]
S2  TL36PO  [TL3XPO]
S4  TL36PO  [TL3XPO]
SW3  SW-C10  [SW-C10]
U$1  AT28C256-28DIP  [DIL28-6]
U$2  AT28C256-28DIP  [DIL28-6]
U$3  AT28C256-28DIP  [DIL28-6]
U$4  AT28C256-28DIP  [DIL28-6]
U$5  AT28C256-28DIP  [DIL28-6]
U$6  AT28C256-28DIP  [DIL28-6]
U$7  AT28C256-28DIP  [DIL28-6]
U$8  AT28C256-28DIP  [DIL28-6]
U$9  AT28C256-28DIP  [DIL28-6]
U$10  AT28C256-28DIP  [DIL28-6]
U$11  AT28C256-28DIP  [DIL28-6]
U$12  AT28C256-28DIP  [DIL28-6]

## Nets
45435: IC18.5(B:I1) IC70.4(D0) IC81.5(B:I1) IC155.7(1Y)
345345: IC70.2(D2) IC72.4(B:I0) IC156.7(1Y)
634354: IC18.4(B:I0) IC70.3(D1) IC155.9(2Y)
654654: IC122.7(A6) IC227.16(Q7)
4654654: IC70.1(D3) IC72.5(B:I1) IC156.9(2Y)
5434534: IC122.6(A5) IC227.15(Q6)
AD7: IC302.11(Y8)
AD8: IC303.18(Y1)
AD15: IC303.11(Y8)
AD16: IC28.18(Y1)
AD17: IC28.17(Y2)
AD18: IC28.16(Y3)
AD19: IC28.15(Y4)
ADDR_OFFSET_SRC: IC268.1(!A!/B) IC278.1(!A!/B)
ADDR_SEGMENT_SRC_0: IC273.14(A) IC274.14(A) IC275.14(A) IC276.14(A) IC279.14(A) IC280.14(A) IC281.14(A) IC282.14(A)
ADDR_SEGMENT_SRC_1: IC273.2(B) IC274.2(B) IC275.2(B) IC276.2(B) IC279.2(B) IC280.2(B) IC281.2(B) IC282.2(B)
AH_OUT: IC102.1(G1) IC102.19(G2)
AH_WRT: IC123.1(G)
AL_OUT: IC117.1(G1) IC117.19(G2)
AL_WRT: IC1.1(G)
ALU_0: IC14.9(F0) IC257.2(1A)
ALU_1: IC14.10(F1) IC257.5(2A)
ALU_2: IC14.11(F2) IC257.11(3A)
ALU_3: IC14.13(F3) IC257.14(4A)
ALU_4: IC15.9(F0) IC258.2(1A)
ALU_5: IC15.10(F1) IC258.5(2A)
ALU_6: IC15.11(F2) IC258.11(3A)
ALU_7: IC15.13(F3) IC257.3(1B) IC257.6(2B) IC257.10(3B) IC257.13(4B) IC258.3(1B) IC258.6(2B) IC258.10(3B) IC258.13(4B) IC258.14(4A)
ALU_CF_IN_SRC0: IC167.1(!A!/B)
ALU_CF_IN_SRC1: IC56.14(A)
ALU_CF_IN_SRC2: IC56.2(B)
ALU_CF_OUT_INV: IC58.1(A:I0)
ALU_FINAL_CF: IC58.3(A:O) IC126.4(2D) IC155.12(2C2) IC243.5(1C1)
ALU_MODE: IC14.8(M) IC15.8(M)
ALU_OP0: IC14.6(S0) IC15.6(S0) IC131.3(A:I1) IC138.13(A:I2)
ALU_OP1: IC14.5(S1) IC15.5(S1) IC65.2(A:I0) IC141.13(A:I2)
ALU_OP2: IC14.4(S2) IC15.4(S2) IC65.3(A:I1) IC141.1(A:I0)
ALU_OP3: IC14.3(S3) IC15.3(S3) IC131.2(A:I0) IC138.2(A:I1)
ALU_OUT_SRC: IC257.1(!A!/B) IC258.1(!A!/B)
AUX_FLAGS_OUT: IC116.1(G1) IC116.19(G2)
AUX_FLAGS_WRT: IC128.1(M) IC128.2(N) IC144.1(M) IC144.2(N)
BH_OUT: IC3.1(G1) IC3.19(G2)
BH_WRT: IC153.1(G)
BL_OUT: IC9.1(G1) IC9.19(G2)
BL_WRT: IC100.1(G)
BPH_OUT: IC114.1(G1)
BPH_WRT: IC99.1(G)
BPL_OUT: IC113.1(G1)
BPL_WRT: IC98.1(G)
CF: IC122.3(A2) IC155.10(2C0) IC167.2(1A) IC227.5(Q2) IC243.6(1C0)
CF_FROM_ALU: IC15.16(CN+4) IC58.2(A:I1)
CF_FROM_SHR_MACHINE: IC93.2(1Q) IC103.2(A1) IC243.4(1C2)
CF_IN_SRC_0: IC243.14(A)
CF_IN_SRC_1: IC243.2(B)
CH_OUT: IC146.1(G1) IC146.19(G2)
CH_WRT: IC185.1(G)
CL_OUT: IC2.1(G1) IC2.19(G2)
CL_WRT: IC101.1(G)
CLK: IC7.11(CLK) IC57.4(B:O) IC60.11(CLK) IC61.11(CLK) IC62.11(CLK) IC75.11(CLK) IC76.11(CLK) IC77.11(CLK) IC78.11(CLK) IC79.11(CLK) IC128.7(CLK) IC134.11(CLK) IC135.11(CLK) IC136.11(CLK) IC137.11(CLK) IC139.14(D1) IC144.7(CLK) IC162.11(CLK) IC189.11(CLK) IC204.3(A:CLK) IC248.7(CLK) IC249.7(CLK)
COND_0: IC70.11(A)
COND_1: IC70.10(B)
COND_2: IC70.9(C)
COND_SRC_0: IC155.14(A) IC156.14(A)
COND_SRC_1: IC155.2(B) IC156.2(B)
CONDITION: IC70.5(Y) IC74.5(B:I1)
CS_H_0: IC275.6(1C0)
CS_H_1: IC275.10(2C0)
CS_H_2: IC276.6(1C0)
CS_H_3: IC276.10(2C0)
CS_H_4: IC273.6(1C0)
CS_H_5: IC273.10(2C0)
CS_H_6: IC274.6(1C0)
CS_H_7: IC274.10(2C0)
CS_H_OUT: IC140.1(G1) IC140.19(G2)
CS_H_WRT: IC173.1(G)
CS_L_0: IC282.6(1C0)
CS_L_1: IC282.10(2C0)
CS_L_2: IC279.6(1C0)
CS_L_3: IC279.10(2C0)
CS_L_4: IC280.6(1C0)
CS_L_5: IC280.10(2C0)
CS_L_6: IC281.6(1C0)
CS_L_7: IC281.10(2C0)
CS_L_OUT: IC210.1(G1) IC210.19(G2)
CS_L_WRT: IC205.1(G)
DATA0: IC118.3(1D) IC169.3(1D) IC179.18(A:Y1) IC295.18(A:Y1)
DATA1: IC118.4(2D) IC169.4(2D) IC179.16(A:Y2) IC295.16(A:Y2)
DATA2: IC169.7(3D) IC179.14(A:Y3) IC295.14(A:Y3)
DATA3: IC169.8(4D) IC179.12(A:Y4) IC295.12(A:Y4)
DATA4: IC169.13(5D) IC178.18(A:Y1) IC294.18(A:Y1)
DATA5: IC169.14(6D) IC178.16(A:Y2) IC294.16(A:Y2)
DATA6: IC169.17(7D) IC178.14(A:Y3) IC294.14(A:Y3)
DATA7: IC169.18(8D) IC178.12(A:Y4) IC294.12(A:Y4)
DH_OUT: IC145.1(G1) IC145.19(G2)
DH_WRT: IC184.1(G)
DI_H_OUT: IC267.1(G1) IC267.19(G2)
DI_H_WRT: IC254.1(G)
DI_L_OUT: IC266.1(G1) IC266.19(G2)
DI_L_WRT: IC265.1(G)
DIR: IC116.8(A7) IC128.5(Q3)
DL_OUT: IC245.1(G1) IC245.19(G2)
DMA_ACK: IC116.2(A1) IC144.3(Q1)
DMA_REQ: IC269.3(A:O)
DMA_TRISTATE: IC116.3(A2) IC144.4(Q2) IC250.4(B:I0)
DS_H_0: IC275.5(1C1)
DS_H_1: IC275.11(2C1)
DS_H_2: IC276.5(1C1)
DS_H_3: IC276.11(2C1)
DS_H_4: IC273.5(1C1)
DS_H_5: IC273.11(2C1)
DS_H_6: IC274.5(1C1)
DS_H_7: IC274.11(2C1)
DS_H_OUT: IC215.1(G1) IC215.19(G2)
DS_H_WRT: IC165.1(G)
DS_L_0: IC282.5(1C1)
DS_L_1: IC282.11(2C1)
DS_L_2: IC279.5(1C1)
DS_L_3: IC279.11(2C1)
DS_L_4: IC280.5(1C1)
DS_L_5: IC280.11(2C1)
DS_L_6: IC281.5(1C1)
DS_L_7: IC281.11(2C1)
DS_L_OUT: IC171.1(G1) IC171.19(G2)
DS_L_WRT: IC166.1(G)
ENCODED_INT_STATUS_OUT: IC154.1(G1) IC154.19(G2)
ES_H_0: IC275.3(1C3)
ES_H_1: IC275.13(2C3)
ES_H_2: IC276.3(1C3)
ES_H_3: IC276.13(2C3)
ES_H_4: IC273.3(1C3)
ES_H_5: IC273.13(2C3)
ES_H_6: IC274.3(1C3)
ES_H_7: IC274.13(2C3)
ES_H_OUT: IC264.1(G1) IC264.19(G2)
ES_H_WRT: IC261.1(G)
ES_L_0: IC282.3(1C3)
ES_L_1: IC282.13(2C3)
ES_L_2: IC279.3(1C3)
ES_L_3: IC279.13(2C3)
ES_L_4: IC280.3(1C3)
ES_L_5: IC280.13(2C3)
ES_L_6: IC281.3(1C3)
ES_L_7: IC281.13(2C3)
ES_L_OUT: IC263.1(G1) IC263.19(G2)
ES_L_WRT: IC262.1(G)
FINAL_CONDITION: IC74.6(B:O) IC83.3(B:I)
FINAL_MEM_IO: IC69.5(B:Y3) RN4.14
FINAL_RD: IC69.9(B:Y1) RN4.16
FINAL_WR: IC69.7(B:Y2) RN4.15
FLAGS_REG_OUT: IC122.1(G1) IC122.19(G2)
GND: IC22.15(G) IC23.15(G) IC49.5(2A) IC49.11(3A) IC49.14(4A) IC49.15(G) IC50.7(C0) IC53.11(B4) IC53.12(A4) IC53.14(A3) IC53.15(B3) IC55.2(1A) IC55.5(2A) IC55.11(3A) IC55.14(4A) IC55.15(G) IC56.1(1G) IC56.6(1C0) IC56.15(2G) IC63.2(1A) IC63.5(2A) IC63.11(3A) IC63.14(4A) IC63.15(G) IC68.2(1A) IC68.5(2A) IC68.10(3B) IC68.11(3A) IC68.13(4B) IC68.14(4A) IC68.15(G) IC69.17(B:A4) IC70.7(G) IC73.3(D1) IC94.15(G) IC95.15(G) IC96.15(G) IC97.15(G) IC115.2(A1) IC115.3(A2) IC115.4(A3) IC115.5(A4) IC115.6(A5) IC115.7(A6) IC115.8(A7) IC115.9(A8) IC121.15(G) IC128.9(G1) IC128.10(G2) IC129.3(D1) IC139.9(G1) IC139.10(G2) IC142.3(D1) IC144.9(G1) IC144.10(G2) IC154.2(A1) IC154.3(A2) IC154.4(A3) IC154.8(A7) IC154.9(A8) IC155.1(1G) IC155.15(2G) IC156.1(1G) IC156.15(2G) IC159.3(D1) IC160.3(D1) IC167.15(G) IC186.3(D1) IC199.13(A:I4) IC208.4(1C2) IC226.5(EI) IC227.14(D6) IC227.17(D7) IC227.18(D8) IC248.9(G1) IC248.10(G2) IC249.9(G1) IC249.10(G2) IC255.4(1C2) IC256.4(1C2) IC258.15(G) IC285.3(A2) IC285.5(A1) IC285.7(C0) IC285.12(A4) IC285.14(A3) IC287.2(B2) IC287.6(B1) IC287.11(B4) IC287.15(B3) R5.1 R6.1 R7.1 R8.1 R10.1 R11.1 R12.1 R13.1 R14.1 RN1.9 RN1.10 RN1.11 RN1.12 RN1.13 RN1.14 RN1.15 RN1.16 RN2.9 RN2.10 RN2.11 RN2.12 RN2.13 RN2.14 RN2.15 RN2.16 RN3.9 RN3.10 RN3.11 RN3.12 RN3.13 RN3.14 RN3.15 RN3.16 S1.2(P) S2.3(S) S4.3(S) U$1.1(A14) U$1.14(GND) U$1.20(/CE) U$1.22(/OE) U$1.27(/WE) U$2.1(A14) U$2.14(GND) U$2.20(/CE) U$2.22(/OE) U$2.27(/WE) U$3.1(A14) U$3.14(GND) U$3.20(/CE) U$3.22(/OE) U$3.27(/WE) U$4.1(A14) U$4.14(GND) U$4.20(/CE) U$4.22(/OE) U$4.27(/WE) U$5.1(A14) U$5.14(GND) U$5.20(/CE) U$5.22(/OE) U$5.27(/WE) U$6.1(A14) U$6.14(GND) U$6.20(/CE) U$6.22(/OE) U$6.27(/WE) U$7.1(A14) U$7.14(GND) U$7.20(/CE) U$7.22(/OE) U$7.27(/WE) U$8.1(A14) U$8.14(GND) U$8.20(/CE) U$8.22(/OE) U$8.27(/WE) U$9.1(A14) U$9.14(GND) U$9.20(/CE) U$9.22(/OE) U$9.27(/WE)
HALT: IC116.7(A6) IC128.4(Q2) IC147.5(B:I1)
IMM_X_OUT: IC115.1(G1) IC115.19(G2)
IMMY_OUT: IC19.1(G1) IC19.19(G2)
IN_TRAP: IC116.6(A5) IC128.3(Q1) IC270.3(B:I) IC271.3(B:I)
INT_ACK: IC222.4(G2A) IC222.5(G2B)
INT_ENABLE: IC64.2(A:I1) IC116.4(A3) IC132.2(A:I1) IC144.5(Q3) IC150.2(A:I1) IC151.2(A:I1) IC157.2(A:I1) IC158.2(A:I1) IC191.2(A:I1)
INT_PENDING: IC141.6(B:O)
INT_REQ_1: IC163.3(A:CLK) R6.2
INT_REQ_2: IC164.3(A:CLK) R7.2
INT_REQ_3: IC168.3(A:CLK) R8.2
INT_REQ_4: IC174.3(A:CLK) R10.2
INT_REQ_5: IC188.3(A:CLK) R11.2
INT_REQ_6: IC221.3(A:CLK) R12.2
INT_REQ_7: IC187.3(A:CLK) R13.2
INTERRUPT_STATUS_OUT: IC125.1(G1) IC125.19(G2)
IO_DMA_REQ: IC204.2(A:D) R14.2
IR_0: IC34.3(D1) IC169.2(1Q)
IR_1: IC35.3(D1)
IR_2: IC36.3(D1)
IR_3: IC37.3(D1)
IR_4: IC38.3(D1)
IR_5: IC40.3(D1)
IR_6: IC41.3(D1)
IR_7: IC71.3(D1) IC169.19(8Q)
IR_8: IC20.3(D1) IC118.2(1Q)
IR_9: IC118.5(2Q) IC172.3(D1)
IR_H_WRT: IC118.1(G)
IR_L_WRT: IC169.1(G)
MAR_H_0: IC277.2(1A)
MAR_H_1: IC277.5(2A)
MAR_H_2: IC277.11(3A)
MAR_H_3: IC277.14(4A)
MAR_H_4: IC278.2(1A)
MAR_H_5: IC278.5(2A)
MAR_H_6: IC278.11(3A)
MAR_H_7: IC278.14(4A)
MAR_L_0: IC268.2(1A)
MAR_L_1: IC268.5(2A)
MAR_L_2: IC268.11(3A)
MAR_L_3: IC268.14(4A)
MAR_L_4: IC272.2(1A)
MAR_L_5: IC272.5(2A)
MAR_L_6: IC272.11(3A)
MAR_L_7: IC272.14(4A)
MARH_WRT: IC7.1(G)
MARH_X_OUT: IC24.19(B:G) IC25.19(B:G)
MARL_0: IC27.11(B:A1) IC189.2(1Q)
MARL_1: IC27.13(B:A2) IC189.5(2Q)
MARL_WRT: IC189.1(G)
MARL_X_OUT: IC26.19(B:G) IC27.19(B:G)
MASK_0: IC244.11(B:A1) IC248.3(Q1)
MASK_1: IC152.9(C:I0) IC244.13(B:A2) IC248.4(Q2)
MASK_2: IC201.9(C:I0) IC244.15(B:A3) IC248.5(Q3)
MASK_3: IC203.9(C:I0) IC244.17(B:A4) IC248.6(Q4)
MASK_4: IC206.9(C:I0) IC247.11(B:A1) IC249.3(Q1)
MASK_5: IC228.9(C:I0) IC247.13(B:A2) IC249.4(Q2)
MASK_6: IC190.9(C:I0) IC247.15(B:A3) IC249.5(Q3)
MASK_7: IC242.9(C:I0)
MASK_ENABLE: IC116.5(A4) IC144.6(Q4) IC152.10(C:I1) IC190.10(C:I1) IC201.10(C:I1) IC203.10(C:I1) IC206.10(C:I1) IC228.10(C:I1) IC242.10(C:I1)
MASK_FLAGS_OUT: IC244.19(B:G) IC247.19(B:G)
MASK_FLAGS_WRT: IC248.1(M) IC248.2(N) IC249.1(M) IC249.2(N)
MDR_IN_BUS0: IC21.3(1D) IC180.3(1D)
MDR_IN_BUS1: IC21.4(2D) IC180.4(2D)
MDR_IN_BUS2: IC21.7(3D) IC180.7(3D)
MDR_IN_BUS3: IC21.8(4D) IC180.8(4D)
MDR_IN_BUS4: IC21.13(5D) IC180.13(5D)
MDR_IN_BUS5: IC21.14(6D) IC180.14(6D)
MDR_IN_BUS6: IC21.17(7D) IC180.17(7D)
MDR_IN_BUS7: IC21.18(8D) IC180.18(8D)
MDR_IN_BUS8: IC296.3(1D) IC301.3(1D)
MDR_IN_BUS9: IC296.4(2D) IC301.4(2D)
MDR_IN_BUS10: IC296.7(3D) IC301.7(3D)
MDR_IN_BUS11: IC296.8(4D) IC301.8(4D)
MDR_IN_BUS12: IC296.13(5D) IC301.13(5D)
MDR_IN_BUS13: IC296.14(6D) IC301.14(6D)
MDR_IN_BUS14: IC296.17(7D) IC301.17(7D)
MDR_IN_BUS15: IC296.18(8D) IC301.18(8D)
MDR_IN_SRC: IC22.1(!A!/B) IC23.1(!A!/B)
MDRH_H_DATA_OUT: IC294.1(A:G) IC295.1(A:G)
MDRH_H_WRT: IC296.1(G)
MDRH_H_X_OUT: IC297.1(A:G) IC298.1(A:G)
MDRH_H_Y_OUT: IC299.1(A:G) IC300.1(A:G)
MDRH_L_DATA_OUT: IC292.1(A:G) IC293.1(A:G)
MDRH_L_WRT: IC301.1(G)
MDRH_L_X_OUT: IC290.1(A:G) IC291.1(A:G)
MDRH_L_Y_OUT: IC288.1(A:G) IC289.1(A:G)
MDRL_H_DATA_OUT: IC178.1(A:G) IC179.1(A:G)
MDRL_H_WRT: IC180.1(G)
MDRL_H_X_OUT: IC176.1(A:G) IC181.1(A:G)
MDRL_H_Y_OUT: IC182.1(A:G) IC183.1(A:G)
MDRL_L_DATA_OUT: IC30.1(A:G) IC31.1(A:G)
MDRL_L_WRT: IC21.1(G)
MDRL_L_X_OUT: IC12.1(A:G) IC13.1(A:G)
MDRL_L_Y_OUT: IC10.1(A:G) IC11.1(A:G)
MEM_IO: IC60.6(Q3) IC69.15(B:A3)
N$1: IC1.2(1Q) IC117.2(A1)
N$2: IC1.5(2Q) IC117.3(A2)
N$3: IC1.6(3Q) IC117.4(A3)
N$4: IC1.9(4Q) IC117.5(A4)
N$5: IC1.12(5Q) IC117.6(A5)
N$6: IC1.15(6Q) IC117.7(A6)
N$7: IC102.8(A7) IC123.16(7Q)
N$8: IC1.19(8Q) IC117.9(A8)
N$9: IC139.1(M) IC139.2(N) IC147.6(B:O)
N$10: IC80.6(B:O) IC133.2(A:I1)
N$11: IC82.19(8Q) IC95.10(3B) IC104.9(A8) IC161.1(A:I0)
N$12: IC49.4(1Y) IC50.6(B1)
N$13: IC9.2(A1) IC100.2(1Q)
N$14: IC49.7(2Y) IC50.2(B2)
N$15: IC9.3(A2) IC100.5(2Q)
N$16: IC9.4(A3) IC100.6(3Q)
N$17: IC9.5(A4) IC100.9(4Q)
N$18: IC9.6(A5) IC100.12(5Q)
N$19: IC9.7(A6) IC100.15(6Q)
N$20: IC9.8(A7) IC100.16(7Q)
N$21: IC9.9(A8) IC100.19(8Q)
N$22: IC56.3(1C3) IC57.2(A:O)
N$23: IC65.1(A:O) IC138.1(A:I0)
N$24: IC143.3(A:O) IC170.5(B:I1)
N$25: IC2.2(A1) IC101.2(1Q)
N$26: IC2.3(A2) IC101.5(2Q)
N$27: IC2.4(A3) IC101.6(3Q)
N$28: IC2.5(A4) IC101.9(4Q)
N$29: IC2.6(A5) IC101.12(5Q)
N$30: IC2.7(A6) IC101.15(6Q)
N$31: IC2.8(A7) IC101.16(7Q)
N$32: IC2.9(A8) IC101.19(8Q)
N$33: IC56.4(1C2) IC57.1(A:I) IC167.4(1Y)
N$34: IC131.1(A:O) IC141.2(A:I1)
N$35: IC49.9(3Y) IC50.15(B3)
N$36: IC49.12(4Y) IC50.11(B4)
N$37: IC51.6(B1) IC55.4(1Y)
N$38: IC51.2(B2) IC55.7(2Y)
N$39: IC51.15(B3) IC55.9(3Y)
N$40: IC51.11(B4) IC55.12(4Y)
N$41: IC227.3(D1) IC241.7(1Y)
N$42: IC179.2(A:A1) IC180.2(1Q) IC181.2(A:A1) IC182.2(A:A1)
N$43: IC179.4(A:A2) IC180.5(2Q) IC181.4(A:A2) IC182.4(A:A2)
N$44: IC179.6(A:A3) IC180.6(3Q) IC181.6(A:A3) IC182.6(A:A3)
N$45: IC179.8(A:A4) IC180.9(4Q) IC181.8(A:A4) IC182.8(A:A4)
N$46: IC176.2(A:A1) IC178.2(A:A1) IC180.12(5Q) IC183.2(A:A1)
N$47: IC176.4(A:A2) IC178.4(A:A2) IC180.15(6Q) IC183.4(A:A2)
N$48: IC176.6(A:A3) IC178.6(A:A3) IC180.16(7Q) IC183.6(A:A3)
N$49: IC204.5(A:Q) IC269.1(A:I0)
N$50: IC66.2(A:I0) IC130.6(B:O) IC143.2(A:I1)
N$51: IC176.8(A:A4) IC178.8(A:A4) IC180.19(8Q) IC183.8(A:A4)
N$52: IC27.15(B:A3) IC189.6(3Q)
N$53: IC27.17(B:A4) IC189.9(4Q)
N$54: IC26.11(B:A1) IC189.12(5Q)
N$55: IC26.13(B:A2) IC189.15(6Q)
N$56: IC26.15(B:A3) IC189.16(7Q)
N$57: IC26.17(B:A4) IC189.19(8Q)
N$58: IC7.2(1Q) IC25.11(B:A1)
N$59: IC7.5(2Q) IC25.13(B:A2)
N$60: IC7.6(3Q) IC25.15(B:A3)
N$61: IC7.9(4Q) IC25.17(B:A4)
N$62: IC7.12(5Q) IC24.11(B:A1)
N$63: IC7.15(6Q) IC24.13(B:A2)
N$64: IC7.16(7Q) IC24.15(B:A3)
N$65: IC52.6(B1) IC63.4(1Y)
N$66: IC122.8(A7) IC227.19(Q8)
N$67: IC5.2(1Q) IC109.11(B:A1)
N$68: IC5.5(2Q) IC109.13(B:A2)
N$69: IC5.6(3Q) IC109.15(B:A3)
N$70: IC5.9(4Q) IC109.17(B:A4)
N$71: IC5.12(5Q) IC110.11(B:A1)
N$72: IC5.15(6Q) IC110.13(B:A2)
N$73: IC7.19(8Q) IC24.17(B:A4)
N$74: IC52.2(B2) IC63.7(2Y)
N$75: IC52.15(B3) IC63.9(3Y)
N$76: IC44.3(A:CLK) IC139.7(CLK) SW3.C
N$77: IC75.3(D1) U$1.11(I/O0)
N$78: IC39.1(A:I0) IC43.4(B:O) IC45.1(A:I0)
N$79: IC32.3(D1) IC186.5(Y)
N$80: IC83.4(B:O) IC85.13(A:I2)
N$81: IC82.2(1Q) IC94.13(4B) IC104.2(A1)
N$82: IC66.1(A:O) IC170.4(B:I0)
N$83: IC10.2(A:A1) IC13.2(A:A1) IC21.2(1Q) IC30.2(A:A1)
N$84: IC133.1(A:I0) IC170.6(B:O)
N$85: IC66.3(A:I1) IC138.12(A:O)
N$86: IC59.1(A:I) IC209.6(B:O)
N$87: IC145.2(A1) IC184.2(1Q)
N$88: IC227.4(D2) IC243.7(1Y)
N$89: IC141.12(A:O) IC143.1(A:I0)
N$90: IC227.7(D3) IC255.7(1Y)
N$91: IC46.5(B:I1) IC47.3(A:O)
N$92: IC227.8(D4) IC256.7(1Y)
N$93: IC208.7(1Y) IC227.13(D5)
N$94: IC46.4(B:I0) IC119.4(B:O)
N$95: IC46.6(B:O) IC124.2(A:I1)
N$96: IC124.3(A:O) IC126.3(1D)
N$97: IC32.4(D2) IC160.5(Y)
N$98: IC257.4(1Y) RN5.16
N$99: IC257.7(2Y) RN5.15
N$100: IC257.9(3Y) RN5.14
N$101: IC257.12(4Y) RN5.13
N$102: IC258.4(1Y) RN5.12
N$103: IC258.7(2Y) RN5.11
N$104: IC258.9(3Y) RN5.10
N$105: IC258.12(4Y) RN5.9
N$106: IC99.19(8Q) IC114.9(A8)
N$107: IC14.16(CN+4) IC15.7(CN)
N$108: IC95.13(4B) IC161.3(A:O)
N$109: IC145.3(A2) IC184.5(2Q)
N$110: IC1.16(7Q) IC117.8(A7)
N$111: IC145.4(A3) IC184.6(3Q)
N$112: IC145.5(A4) IC184.9(4Q)
N$113: IC32.7(D3) IC159.5(Y)
N$114: IC86.2(1Q) IC89.2(A:A1)
N$115: IC86.5(2Q) IC89.4(A:A2)
N$116: IC86.6(3Q) IC89.6(A:A3)
N$117: IC86.9(4Q) IC89.8(A:A4)
N$118: IC86.12(5Q) IC90.2(A:A1)
N$119: IC86.15(6Q) IC90.4(A:A2)
N$120: IC86.16(7Q) IC90.6(A:A3)
N$121: IC86.19(8Q) IC90.8(A:A4)
N$122: IC88.2(1Q) IC91.2(A:A1)
N$123: IC88.5(2Q) IC91.4(A:A2)
N$124: IC88.6(3Q) IC91.6(A:A3)
N$125: IC88.9(4Q) IC91.8(A:A4)
N$126: IC88.12(5Q) IC92.2(A:A1)
N$127: IC88.15(6Q) IC92.4(A:A2)
N$128: IC88.16(7Q) IC92.6(A:A3)
N$129: IC88.19(8Q) IC92.8(A:A4)
N$130: IC42.2(A:I1) IC67.6(B:O)
N$131: IC93.3(1D) IC96.4(1Y)
N$132: IC10.4(A:A2) IC13.4(A:A2) IC21.5(2Q) IC30.4(A:A2)
N$133: IC45.3(A:O) IC67.5(B:I1)
N$134: IC10.6(A:A3) IC13.6(A:A3) IC21.6(3Q) IC30.6(A:A3)
N$135: IC145.6(A5) IC184.12(5Q)
N$136: IC145.7(A6) IC184.15(6Q)
N$137: IC10.8(A:A4) IC13.8(A:A4) IC21.9(4Q) IC30.8(A:A4)
N$138: IC11.2(A:A1) IC12.2(A:A1) IC21.12(5Q) IC31.2(A:A1)
N$139: IC145.8(A7) IC184.16(7Q)
N$140: IC11.4(A:A2) IC12.4(A:A2) IC21.15(6Q) IC31.4(A:A2)
N$141: IC11.6(A:A3) IC12.6(A:A3) IC21.16(7Q) IC31.6(A:A3)
N$142: IC145.9(A8) IC184.19(8Q)
N$143: IC5.16(7Q) IC110.15(B:A3)
N$144: IC52.11(B4) IC63.12(4Y)
N$145: IC53.6(B1) IC68.4(1Y)
N$146: IC5.19(8Q) IC110.17(B:A4)
N$147: IC53.2(B2) IC68.7(2Y)
N$148: IC93.4(2D) IC96.7(2Y)
N$149: IC93.7(3D) IC96.9(3Y)
N$150: IC55.13(4B) IC63.3(1B) IC63.6(2B) IC63.10(3B) IC63.13(4B) IC68.3(1B) IC68.6(2B)
N$151: IC4.2(1Q) IC111.11(B:A1)
N$152: IC49.1(!A!/B) IC55.1(!A!/B) IC63.1(!A!/B) IC68.1(!A!/B) IC85.12(A:O)
N$153: IC32.8(D4) IC142.5(Y)
N$154: IC84.4(B:O) IC85.2(A:I1)
N$155: IC268.15(G) IC272.15(G) IC277.15(G) IC278.15(G)
N$156: IC93.8(4D) IC96.12(4Y)
N$157: IC93.13(5D) IC94.4(1Y)
N$158: IC93.14(6D) IC94.7(2Y)
N$159: IC93.17(7D) IC94.9(3Y)
N$160: IC93.18(8D) IC94.12(4Y)
N$161: IC82.3(1D) IC97.4(1Y)
N$162: IC82.4(2D) IC97.7(2Y)
N$163: IC82.7(3D) IC97.9(3Y)
N$164: IC11.8(A:A4) IC12.8(A:A4) IC21.19(8Q) IC31.8(A:A4)
N$165: IC82.8(4D) IC97.12(4Y)
N$166: IC82.13(5D) IC95.4(1Y)
N$167: SW3.2
N$168: IC82.14(6D) IC95.7(2Y)
N$169: IC10.18(A:Y1)
N$170: IC10.16(A:Y2)
N$171: IC10.14(A:Y3)
N$172: IC10.12(A:Y4)
N$173: IC82.17(7D) IC95.9(3Y)
N$174: IC32.13(D5) IC129.5(Y)
N$175: IC32.14(D6) IC73.5(Y)
N$176: IC14.7(CN) IC56.7(1Y)
N$177: IC13.18(A:Y1)
N$178: IC13.16(A:Y2)
N$179: IC13.14(A:Y3)
N$180: IC13.12(A:Y4)
N$181: IC12.18(A:Y1)
N$182: IC12.16(A:Y2)
N$183: IC12.14(A:Y3)
N$184: IC12.12(A:Y4)
N$185: IC32.17(D7) IC34.5(Y)
N$186: IC32.18(D8) IC35.5(Y)
N$187: IC33.3(D1) IC36.5(Y)
N$188: IC33.4(D2) IC37.5(Y)
N$189: IC33.7(D3) IC38.5(Y)
N$190: IC33.8(D4) IC40.5(Y)
N$191: IC22.7(2Y)
N$192: IC22.9(3Y)
N$193: IC22.12(4Y)
N$194: IC23.4(1Y)
N$195: IC23.7(2Y)
N$196: IC23.9(3Y)
N$197: IC23.12(4Y)
N$198: IC22.3(1B)
N$199: IC22.6(2B)
N$200: IC30.18(A:Y1)
N$201: IC30.16(A:Y2)
N$202: IC82.18(8D) IC95.12(4Y)
N$203: IC30.14(A:Y3)
N$204: IC30.12(A:Y4)
N$205: IC82.16(7Q) IC95.6(2B) IC104.8(A7)
N$206: IC31.18(A:Y1)
N$207: IC31.16(A:Y2)
N$208: IC31.14(A:Y3)
N$209: IC31.12(A:Y4)
N$210: IC22.4(1Y)
N$211: IC22.10(3B)
N$212: IC22.13(4B)
N$213: IC23.3(1B)
N$214: IC23.6(2B)
N$215: IC23.10(3B)
N$216: IC23.13(4B)
N$217: IC116.9(A8) IC128.6(Q4)
N$218: IC33.13(D5) IC41.5(Y)
N$219: IC33.14(D6) IC71.5(Y)
N$220: IC148.3(A:O) IC162.3(D1)
N$221: IC102.6(A5) IC123.12(5Q)
N$222: IC195.2(A:I1) IC222.15(Y0)
N$223: IC8.1(A:CLR) IC195.3(A:O)
N$224: IC8.5(A:Q) IC148.2(A:I1)
N$225: IC20.5(Y) IC33.17(D7)
N$226: IC196.4(B:O) IC226.4
N$227: IC39.3(A:O)
N$228: IC33.18(D8) IC172.5(Y)
N$229: IC102.7(A6) IC123.15(6Q)
N$230: IC205.2(1Q) IC210.2(A1)
N$231: IC120.3(A:O) IC241.4(1C2)
N$232: IC82.15(6Q) IC95.3(1B) IC104.7(A6)
N$233: IC82.12(5Q) IC97.13(4B) IC104.6(A5)
N$234: IC205.5(2Q) IC210.3(A2)
N$235: IC102.9(A8) IC123.19(8Q)
N$236: IC102.2(A1) IC123.2(1Q)
N$237: IC102.3(A2) IC123.5(2Q)
N$238: IC102.4(A3) IC123.6(3Q)
N$239: IC205.6(3Q) IC210.4(A3)
N$240: IC205.9(4Q) IC210.5(A4)
N$241: IC205.12(5Q) IC210.6(A5)
N$242: IC205.15(6Q) IC210.7(A6)
N$243: IC205.16(7Q) IC210.8(A7)
N$244: IC205.19(8Q) IC210.9(A8)
N$245: IC140.2(A1) IC173.2(1Q)
N$246: IC140.3(A2) IC173.5(2Q)
N$247: IC140.4(A3) IC173.6(3Q)
N$248: IC140.5(A4) IC173.9(4Q)
N$249: IC102.5(A4) IC123.9(4Q)
N$250: IC140.6(A5) IC173.12(5Q)
N$251: U$2.10(A0)
N$252: U$2.9(A1)
N$253: U$2.8(A2)
N$254: U$2.7(A3)
N$255: U$2.6(A4)
N$256: U$2.5(A5)
N$257: U$2.4(A6)
N$258: U$2.3(A7)
N$259: U$2.25(A8)
N$260: U$2.24(A9)
N$261: U$2.21(A10)
N$262: U$2.23(A11)
N$263: U$2.2(A12)
N$264: U$2.26(A13)
N$265: U$3.10(A0)
N$266: U$3.9(A1)
N$267: U$3.8(A2)
N$268: U$3.7(A3)
N$269: U$3.6(A4)
N$270: U$3.5(A5)
N$271: U$3.4(A6)
N$272: U$3.3(A7)
N$273: U$3.25(A8)
N$274: U$3.24(A9)
N$275: U$3.21(A10)
N$276: U$3.23(A11)
N$277: U$3.2(A12)
N$278: U$3.26(A13)
N$279: U$4.10(A0)
N$280: U$4.9(A1)
N$281: U$4.8(A2)
N$282: U$4.7(A3)
N$283: U$4.6(A4)
N$284: U$4.5(A5)
N$285: U$4.4(A6)
N$286: U$4.3(A7)
N$287: U$4.25(A8)
N$288: U$4.24(A9)
N$289: U$4.21(A10)
N$290: U$4.23(A11)
N$291: U$4.2(A12)
N$292: U$4.26(A13)
N$293: U$5.10(A0)
N$294: U$5.9(A1)
N$295: U$5.8(A2)
N$296: U$5.7(A3)
N$297: U$5.6(A4)
N$298: U$5.5(A5)
N$299: U$5.4(A6)
N$300: U$5.3(A7)
N$301: U$5.25(A8)
N$302: U$5.24(A9)
N$303: U$5.21(A10)
N$304: U$5.23(A11)
N$305: U$5.2(A12)
N$306: U$5.26(A13)
N$307: IC140.7(A6) IC173.15(6Q)
N$308: IC140.8(A7) IC173.16(7Q)
N$309: IC140.9(A8) IC173.19(8Q)
N$310: IC166.2(1Q) IC171.2(A1)
N$311: IC166.5(2Q) IC171.3(A2)
N$312: IC82.9(4Q) IC97.10(3B) IC104.5(A4)
N$313: IC82.6(3Q) IC97.6(2B) IC104.4(A3)
N$314: IC82.5(2Q) IC97.3(1B) IC104.3(A2)
N$315: IC166.6(3Q) IC171.4(A3)
N$316: IC93.19(8Q) IC94.10(3B) IC103.9(A8)
N$317: IC93.16(7Q) IC94.6(2B) IC103.8(A7)
N$318: IC93.15(6Q) IC94.3(1B) IC103.7(A6)
N$319: IC93.12(5Q) IC96.13(4B) IC103.6(A5)
N$320: IC154.7(A6) IC226.9(A0)
N$321: IC93.9(4Q) IC96.10(3B) IC103.5(A4)
N$322: IC175.6(B:O) IC177.4(B:I0)
N$323: IC93.6(3Q) IC96.6(2B) IC103.4(A3)
N$324: IC177.6(B:O) IC192.4(B:I0)
N$325: IC3.2(A1) IC153.2(1Q)
N$326: IC3.3(A2) IC153.5(2Q)
N$327: IC3.4(A3) IC153.6(3Q)
N$328: IC3.5(A4) IC153.9(4Q)
N$329: IC3.6(A5) IC153.12(5Q)
N$330: IC3.7(A6) IC153.15(6Q)
N$331: IC3.8(A7) IC153.16(7Q)
N$332: IC3.9(A8) IC153.19(8Q)
N$333: IC50.5(A1)
N$334: IC50.3(A2)
N$335: IC50.14(A3)
N$336: IC50.12(A4)
N$337: IC52.5(A1)
N$338: IC51.5(A1)
N$339: IC51.3(A2)
N$340: IC51.14(A3)
N$341: IC51.12(A4)
N$342: IC146.2(A1) IC185.2(1Q)
N$343: IC93.5(2Q) IC96.3(1B) IC103.3(A2)
N$344: IC166.9(4Q) IC171.5(A4)
N$345: IC166.12(5Q) IC171.6(A5)
N$346: IC158.1(A:I0) IC190.8(C:O)
N$347: IC121.3(1B) IC127.3(A:O)
N$348: IC125.2(A1) IC162.2(Q1) IC196.3(B:I)
N$349: IC149.3(B:I) IC226.14(GS)
N$350: IC52.3(A2)
N$351: IC52.14(A3)
N$352: IC52.12(A4)
N$353: IC53.5(A1)
N$354: IC53.3(A2)
N$355: IC158.12(A:O) IC226.11
N$356: IC141.4(B:I1) IC149.4(B:O)
N$357: IC50.9(C4) IC51.7(C0)
N$358: IC51.9(C4) IC52.7(C0)
N$359: IC52.9(C4) IC53.7(C0)
N$360: IC76.5(Q2)
N$361: IC141.3(B:I0) IC226.15(EO)
N$362: IC192.6(B:O) IC193.4(B:I0)
N$363: IC166.15(6Q) IC171.7(A6)
N$364: IC76.6(Q3)
N$365: IC64.12(A:O) IC226.3
N$366: IC64.13(A:I2) IC125.3(A2) IC162.5(Q2)
N$367: IC75.4(D2) U$1.12(I/O1)
N$368: IC132.1(A:I0) IC201.8(C:O)
N$369: IC75.7(D3) U$1.13(I/O2)
N$370: IC166.16(7Q) IC171.8(A7)
N$371: IC166.19(8Q) IC171.9(A8)
N$372: IC168.1(A:CLR) IC220.3(A:O)
N$373: IC146.3(A2) IC185.5(2Q)
N$374: IC174.1(A:CLR) IC223.3(A:O)
N$375: IC75.8(D4) U$1.15(I/O3)
N$376: IC75.13(D5) U$1.16(I/O4)
N$377: IC75.14(D6) U$1.17(I/O5)
N$378: IC60.3(D1) U$10.11(I/O0)
N$379: IC60.4(D2) U$10.12(I/O1)
N$380: IC60.7(D3) U$10.13(I/O2)
N$381: IC60.8(D4) U$10.15(I/O3)
N$382: IC60.13(D5) U$10.16(I/O4)
N$383: IC60.14(D6) U$10.17(I/O5)
N$384: IC60.17(D7) U$10.18(I/O6)
N$385: IC60.18(D8) U$10.19(I/O7)
N$386: IC61.3(D1) U$11.11(I/O0)
N$387: IC61.4(D2) U$11.12(I/O1)
N$388: IC188.1(A:CLR) IC224.3(A:O)
N$389: IC162.18(D8) IC187.5(A:Q)
N$390: IC162.4(D2) IC163.5(A:Q)
N$391: IC76.9(Q4)
N$392: IC162.7(D3) IC164.5(A:Q)
N$393: IC162.8(D4) IC168.5(A:Q)
N$394: IC162.13(D5) IC174.5(A:Q)
N$395: IC162.14(D6) IC188.5(A:Q)
N$396: IC162.17(D7) IC221.5(A:Q)
N$397: IC207.1(A:I0) IC222.7(Y7)
N$398: IC218.2(A:I1) IC222.14(Y1)
N$399: IC219.2(A:I1) IC222.13(Y2)
N$400: IC76.12(Q5)
N$401: IC76.15(Q6)
N$402: IC76.16(Q7)
N$403: IC222.11(Y4) IC223.1(A:I0)
N$404: IC4.5(2Q) IC111.13(B:A2)
N$405: IC222.9(Y6) IC225.1(A:I0)
N$406: IC187.1(A:CLR) IC207.3(A:O)
N$407: IC251.2(1Q) IC252.2(A1)
N$408: IC163.1(A:CLR) IC218.3(A:O)
N$409: IC164.1(A:CLR) IC219.3(A:O)
N$410: IC221.1(A:CLR) IC225.3(A:O)
N$411: IC125.4(A3) IC132.13(A:I2) IC162.6(Q3)
N$412: IC125.5(A4) IC150.13(A:I2) IC162.9(Q4)
N$413: IC132.12(A:O) IC226.2
N$414: IC125.6(A5) IC151.13(A:I2) IC162.12(Q5)
N$415: IC150.1(A:I0) IC203.8(C:O)
N$416: IC150.12(A:O) IC226.1
N$417: IC151.1(A:I0) IC206.8(C:O)
N$418: IC151.12(A:O) IC226.13
N$419: IC157.1(A:I0) IC228.8(C:O)
N$420: IC157.12(A:O) IC226.12
N$421: IC191.1(A:I0) IC242.8(C:O)
N$422: IC146.4(A3) IC185.6(3Q)
N$423: IC146.5(A4) IC185.9(4Q)
N$424: IC146.6(A5) IC185.12(5Q)
N$425: IC146.7(A6) IC185.15(6Q)
N$426: IC146.8(A7) IC185.16(7Q)
N$427: IC146.9(A8) IC185.19(8Q)
N$428: IC216.2(1Q) IC245.2(A1)
N$429: IC216.5(2Q) IC245.3(A2)
N$430: IC216.6(3Q) IC245.4(A3)
N$431: IC216.9(4Q) IC245.5(A4)
N$432: IC216.12(5Q) IC245.6(A5)
N$433: IC216.15(6Q) IC245.7(A6)
N$434: IC216.16(7Q) IC245.8(A7)
N$435: IC216.19(8Q) IC245.9(A8)
N$436: IC191.12(A:O) IC226.10
N$437: IC125.7(A6) IC157.13(A:I2) IC162.15(Q6)
N$438: IC125.8(A7) IC158.13(A:I2) IC162.16(Q7)
N$439: IC125.9(A8) IC162.19(Q8) IC191.13(A:I2)
N$440: IC76.19(Q8)
N$441: IC165.2(1Q) IC215.2(A1)
N$442: IC76.3(D1) U$2.11(I/O0)
N$443: IC76.4(D2) U$2.12(I/O1)
N$444: IC247.17(B:A4) IC249.6(Q4)
N$445: IC193.6(B:O) IC194.4(B:I0)
N$446: IC197.5(A:O) IC198.1(A:I)
N$447: IC77.5(Q2)
N$448: IC61.7(D3) U$11.13(I/O2)
N$449: IC75.17(D7) U$1.18(I/O6)
N$450: IC75.18(D8) U$1.19(I/O7)
N$451: IC76.7(D3) U$2.13(I/O2)
N$452: IC76.8(D4) U$2.15(I/O3)
N$453: IC76.13(D5) U$2.16(I/O4)
N$454: IC76.14(D6) U$2.17(I/O5)
N$455: IC76.17(D7) U$2.18(I/O6)
N$456: IC76.18(D8) U$2.19(I/O7)
N$457: IC77.3(D1) U$3.11(I/O0)
N$458: IC77.4(D2) U$3.12(I/O1)
N$459: IC77.7(D3) U$3.13(I/O2)
N$460: IC77.8(D4) U$3.15(I/O3)
N$461: IC77.13(D5) U$3.16(I/O4)
N$462: IC77.14(D6) U$3.17(I/O5)
N$463: IC77.17(D7) U$3.18(I/O6)
N$464: IC77.18(D8) U$3.19(I/O7)
N$465: IC78.3(D1) U$4.11(I/O0)
N$466: IC78.4(D2) U$4.12(I/O1)
N$467: IC78.7(D3) U$4.13(I/O2)
N$468: IC78.8(D4) U$4.15(I/O3)
N$469: IC78.13(D5) U$4.16(I/O4)
N$470: IC78.14(D6) U$4.17(I/O5)
N$471: IC78.17(D7) U$4.18(I/O6)
N$472: IC78.18(D8) U$4.19(I/O7)
N$473: IC79.3(D1) U$5.11(I/O0)
N$474: IC79.4(D2) U$5.12(I/O1)
N$475: IC79.7(D3) U$5.13(I/O2)
N$476: IC79.8(D4) U$5.15(I/O3)
N$477: IC79.13(D5) U$5.16(I/O4)
N$478: IC79.14(D6) U$5.17(I/O5)
N$479: IC79.17(D7) U$5.18(I/O6)
N$480: IC79.18(D8) U$5.19(I/O7)
N$481: IC198.2(A:O) IC199.1(A:I0)
N$482: IC61.8(D4) U$11.15(I/O3)
N$483: IC61.13(D5) U$11.16(I/O4)
N$484: IC61.14(D6) U$11.17(I/O5)
N$485: IC61.17(D7) U$11.18(I/O6)
N$486: IC61.18(D8) U$11.19(I/O7)
N$487: IC62.3(D1) U$12.11(I/O0)
N$488: IC62.4(D2) U$12.12(I/O1)
N$489: IC62.7(D3) U$12.13(I/O2)
N$490: IC62.8(D4) U$12.15(I/O3)
N$491: IC62.13(D5) U$12.16(I/O4)
N$492: IC62.14(D6) U$12.17(I/O5)
N$493: IC62.17(D7) U$12.18(I/O6)
N$494: IC62.18(D8) U$12.19(I/O7)
N$495: IC194.6(B:O) IC200.4(B:I0)
N$496: IC200.6(B:O) IC209.4(B:I0)
N$497: IC165.5(2Q) IC215.3(A2)
N$498: IC165.6(3Q) IC215.4(A3)
N$499: IC165.9(4Q) IC215.5(A4)
N$500: IC165.12(5Q) IC215.6(A5)
N$501: IC165.15(6Q) IC215.7(A6)
N$502: IC165.16(7Q) IC215.8(A7)
N$503: IC134.18(D8) U$6.19(I/O7)
N$504: IC134.17(D7) U$6.18(I/O6)
N$505: IC134.14(D6) U$6.17(I/O5)
N$506: IC134.13(D5) U$6.16(I/O4)
N$507: IC134.8(D4) U$6.15(I/O3)
N$508: IC134.7(D3) U$6.13(I/O2)
N$509: IC134.4(D2) U$6.12(I/O1)
N$510: IC134.3(D1) U$6.11(I/O0)
N$511: IC135.3(D1) U$7.11(I/O0)
N$512: IC135.4(D2) U$7.12(I/O1)
N$513: IC135.7(D3) U$7.13(I/O2)
N$514: IC135.8(D4) U$7.15(I/O3)
N$515: IC135.13(D5) U$7.16(I/O4)
N$516: IC135.14(D6) U$7.17(I/O5)
N$517: IC135.17(D7) U$7.18(I/O6)
N$518: IC135.18(D8) U$7.19(I/O7)
N$519: IC136.3(D1) U$8.11(I/O0)
N$520: IC136.4(D2) U$8.12(I/O1)
N$521: IC136.7(D3) U$8.13(I/O2)
N$522: IC136.8(D4) U$8.15(I/O3)
N$523: IC136.13(D5) U$8.16(I/O4)
N$524: IC136.14(D6) U$8.17(I/O5)
N$525: IC136.17(D7) U$8.18(I/O6)
N$526: IC136.18(D8) U$8.19(I/O7)
N$527: IC137.3(D1) U$9.11(I/O0)
N$528: IC87.3(A:S2) R1.1 S1.1(O)
N$529: IC87.1(A:R) R2.1 S1.3(S)
N$530: IC251.5(2Q) IC252.3(A2)
N$531: IC87.4(A:Q) SW3.1
N$532: SW3.4
N$533: IC137.4(D2) U$9.12(I/O1)
N$534: IC137.7(D3) U$9.13(I/O2)
N$535: IC137.8(D4) U$9.15(I/O3)
N$536: IC137.13(D5) U$9.16(I/O4)
N$537: IC137.14(D6) U$9.17(I/O5)
N$538: IC137.17(D7) U$9.18(I/O6)
N$539: IC137.18(D8) U$9.19(I/O7)
N$540: IC251.6(3Q) IC252.4(A3)
N$541: IC64.1(A:I0) IC152.8(C:O)
N$542: IC165.19(8Q) IC215.9(A8)
N$543: IC246.2(1Q) IC259.2(A1)
N$544: IC246.5(2Q) IC259.3(A2)
N$545: IC246.6(3Q) IC259.4(A3)
N$546: IC246.9(4Q) IC259.5(A4)
N$547: IC246.12(5Q) IC259.6(A5)
N$548: IC57.3(B:I) IC139.3(Q1)
N$549: IC246.15(6Q) IC259.7(A6)
N$550: IC246.16(7Q) IC259.8(A7)
N$551: IC246.19(8Q) IC259.9(A8)
N$552: IC217.2(1Q) IC260.2(A1)
N$553: IC217.5(2Q) IC260.3(A2)
N$554: IC217.6(3Q) IC260.4(A3)
N$555: IC217.9(4Q) IC260.5(A4)
N$556: IC217.12(5Q) IC260.6(A5)
N$557: IC217.15(6Q) IC260.7(A6)
N$558: IC217.16(7Q) IC260.8(A7)
N$559: IC217.19(8Q) IC260.9(A8)
N$560: IC262.2(1Q) IC263.2(A1)
N$561: IC262.5(2Q) IC263.3(A2)
N$562: IC262.6(3Q) IC263.4(A3)
N$563: IC262.9(4Q) IC263.5(A4)
N$564: IC77.6(Q3)
N$565: IC262.12(5Q) IC263.6(A5)
N$566: IC262.15(6Q) IC263.7(A6)
N$567: IC70.13(D6) IC81.6(B:O)
N$568: IC77.9(Q4)
N$569: IC18.6(B:O) IC70.12(D7)
N$570: IC262.16(7Q) IC263.8(A7)
N$571: IC77.12(Q5)
N$572: IC262.19(8Q) IC263.9(A8)
N$573: IC261.2(1Q) IC264.2(A1)
N$574: IC16.2(1Q) IC211.2(A:A1)
N$575: IC16.5(2Q) IC211.4(A:A2)
N$576: IC16.6(3Q) IC211.6(A:A3)
N$577: IC4.6(3Q) IC111.15(B:A3)
N$578: IC4.9(4Q) IC111.17(B:A4)
N$579: IC4.12(5Q) IC112.11(B:A1)
N$580: IC4.15(6Q) IC112.13(B:A2)
N$581: IC4.16(7Q) IC112.15(B:A3)
N$582: IC4.19(8Q) IC112.17(B:A4)
N$583: IC98.2(1Q) IC113.2(A1)
N$584: IC98.5(2Q) IC113.3(A2)
N$585: IC98.6(3Q) IC113.4(A3)
N$586: IC98.9(4Q) IC113.5(A4)
N$587: IC98.12(5Q) IC113.6(A5)
N$588: IC98.15(6Q) IC113.7(A6)
N$589: IC98.16(7Q) IC113.8(A7)
N$590: IC98.19(8Q) IC113.9(A8)
N$591: IC99.2(1Q) IC114.2(A1)
N$592: IC99.5(2Q) IC114.3(A2)
N$593: IC99.6(3Q) IC114.4(A3)
N$594: IC99.9(4Q) IC114.5(A4)
N$595: IC99.12(5Q) IC114.6(A5)
N$596: IC99.15(6Q) IC114.7(A6)
N$597: IC99.16(7Q) IC114.8(A7)
N$598: IC261.5(2Q) IC264.3(A2)
N$599: IC261.6(3Q) IC264.4(A3)
N$600: IC261.9(4Q) IC264.5(A4)
N$601: IC16.9(4Q) IC211.8(A:A4)
N$602: IC77.15(Q6)
N$603: IC16.12(5Q) IC212.2(A:A1)
N$604: IC16.15(6Q) IC212.4(A:A2)
N$605: IC77.16(Q7)
N$606: IC77.19(Q8)
N$607: IC261.12(5Q) IC264.6(A5)
N$608: IC261.15(6Q) IC264.7(A6)
N$609: IC261.16(7Q) IC264.8(A7)
N$610: IC261.19(8Q) IC264.9(A8)
N$611: IC251.9(4Q) IC252.5(A4)
N$612: IC251.12(5Q) IC252.6(A5)
N$613: IC251.15(6Q) IC252.7(A6)
N$614: IC251.16(7Q) IC252.8(A7)
N$615: IC251.19(8Q) IC252.9(A8)
N$616: IC202.2(1Q) IC253.2(A1)
N$617: IC202.5(2Q) IC253.3(A2)
N$618: IC202.6(3Q) IC253.4(A3)
N$619: IC202.9(4Q) IC253.5(A4)
N$620: IC202.12(5Q) IC253.6(A5)
N$621: IC202.15(6Q) IC253.7(A6)
N$622: IC202.16(7Q) IC253.8(A7)
N$623: IC202.19(8Q) IC253.9(A8)
N$624: IC265.2(1Q) IC266.2(A1)
N$625: IC265.5(2Q) IC266.3(A2)
N$626: IC265.6(3Q) IC266.4(A3)
N$627: IC265.9(4Q) IC266.5(A4)
N$628: IC265.12(5Q) IC266.6(A5)
N$629: IC265.15(6Q) IC266.7(A6)
N$630: IC265.16(7Q) IC266.8(A7)
N$631: IC265.19(8Q) IC266.9(A8)
N$632: IC254.2(1Q) IC267.2(A1)
N$633: IC254.5(2Q) IC267.3(A2)
N$634: IC254.6(3Q) IC267.4(A3)
N$635: IC254.9(4Q) IC267.5(A4)
N$636: IC254.12(5Q) IC267.6(A5)
N$637: IC254.15(6Q) IC267.7(A6)
N$638: IC254.16(7Q) IC267.8(A7)
N$639: IC254.19(8Q) IC267.9(A8)
N$640: IC141.5(B:I2) IC270.4(B:O)
N$641: IC269.2(A:I1) IC271.4(B:O)
N$642: IC273.1(1G) IC273.15(2G) IC274.1(1G) IC274.15(2G) IC275.1(1G) IC275.15(2G) IC276.1(1G) IC276.15(2G) IC279.1(1G) IC279.15(2G) IC280.1(1G) IC280.15(2G) IC281.1(1G) IC281.15(2G) IC282.1(1G) IC282.15(2G)
N$643: IC268.4(1Y) IC285.6(B1)
N$644: IC268.7(2Y) IC285.2(B2)
N$645: IC268.9(3Y) IC285.15(B3)
N$646: IC268.12(4Y) IC285.11(B4)
N$647: IC272.4(1Y) IC283.6(B1)
N$648: IC272.7(2Y) IC283.2(B2)
N$649: IC272.9(3Y) IC283.15(B3)
N$650: IC272.12(4Y) IC283.11(B4)
N$651: IC277.4(1Y) IC284.6(B1)
N$652: IC277.7(2Y) IC284.2(B2)
N$653: IC277.9(3Y) IC284.15(B3)
N$654: IC277.12(4Y) IC284.11(B4)
N$655: IC16.16(7Q) IC212.6(A:A3)
N$656: IC16.19(8Q) IC212.8(A:A4)
N$657: IC17.2(1Q) IC213.2(A:A1)
N$658: IC17.5(2Q) IC213.4(A:A2)
N$659: IC17.6(3Q) IC213.6(A:A3)
N$660: IC17.9(4Q) IC213.8(A:A4)
N$661: IC17.12(5Q) IC214.2(A:A1)
N$662: IC17.15(6Q) IC214.4(A:A2)
N$663: IC17.16(7Q) IC214.6(A:A3)
N$664: IC17.19(8Q) IC214.8(A:A4)
N$665: IC278.4(1Y) IC286.6(B1)
N$666: IC278.7(2Y) IC286.2(B2)
N$667: IC278.9(3Y) IC286.15(B3)
N$668: IC278.12(4Y) IC286.11(B4)
N$669: IC282.7(1Y) IC283.5(A1)
N$670: IC283.7(C0) IC285.9(C4)
N$671: IC283.9(C4) IC284.7(C0)
N$672: IC284.9(C4) IC286.7(C0)
N$673: IC286.9(C4) IC287.7(C0)
N$674: IC282.9(2Y) IC283.3(A2)
N$675: IC279.7(1Y) IC283.14(A3)
N$676: IC279.9(2Y) IC283.12(A4)
N$677: IC280.7(1Y) IC284.5(A1)
N$678: IC280.9(2Y) IC284.3(A2)
N$679: IC281.7(1Y) IC284.14(A3)
N$680: IC281.9(2Y) IC284.12(A4)
N$681: IC275.7(1Y) IC286.5(A1)
N$682: IC275.9(2Y) IC286.3(A2)
N$683: IC276.7(1Y) IC286.14(A3)
N$684: IC276.9(2Y) IC286.12(A4)
N$685: IC220.1(A:I0) IC222.12(Y3)
N$686: IC273.7(1Y) IC287.5(A1)
N$687: IC222.10(Y5) IC224.1(A:I0)
N$688: IC229.2(A:A1) IC234.2(1Q)
N$689: IC229.4(A:A2) IC234.5(2Q)
N$690: IC229.6(A:A3) IC234.6(3Q)
N$691: IC230.2(A:A1) IC234.12(5Q)
N$692: IC230.4(A:A2) IC234.15(6Q)
N$693: IC230.6(A:A3) IC234.16(7Q)
N$694: IC230.8(A:A4) IC234.19(8Q)
N$695: IC231.2(A:A1) IC233.2(1Q)
N$696: IC231.4(A:A2) IC233.5(2Q)
N$697: IC231.6(A:A3) IC233.6(3Q)
N$698: IC231.8(A:A4) IC233.9(4Q)
N$699: IC232.2(A:A1) IC233.12(5Q)
N$700: IC232.4(A:A2) IC233.15(6Q)
N$701: IC232.6(A:A3) IC233.16(7Q)
N$702: IC232.8(A:A4) IC233.19(8Q)
N$703: IC230.1(A:G)
N$704: IC234.9(4Q)
N$705: IC235.2(A:A1) IC240.2(1Q)
N$706: IC235.4(A:A2) IC240.5(2Q)
N$707: IC235.6(A:A3) IC240.6(3Q)
N$708: IC236.2(A:A1) IC240.12(5Q)
N$709: IC236.4(A:A2) IC240.15(6Q)
N$710: IC236.6(A:A3) IC240.16(7Q)
N$711: IC236.8(A:A4) IC240.19(8Q)
N$712: IC237.2(A:A1) IC239.2(1Q)
N$713: IC237.4(A:A2) IC239.5(2Q)
N$714: IC237.6(A:A3) IC239.6(3Q)
N$715: IC237.8(A:A4) IC239.9(4Q)
N$716: IC238.2(A:A1) IC239.12(5Q)
N$717: IC238.4(A:A2) IC239.15(6Q)
N$718: IC238.6(A:A3) IC239.16(7Q)
N$719: IC238.8(A:A4) IC239.19(8Q)
N$720: IC236.1(A:G)
N$721: IC240.9(4Q)
N$722: IC273.9(2Y) IC287.3(A2)
N$723: IC274.7(1Y) IC287.14(A3)
N$724: IC274.9(2Y) IC287.12(A4)
N$725: IC288.18(A:Y1)
N$726: IC288.16(A:Y2)
N$727: IC288.14(A:Y3)
N$728: IC288.12(A:Y4)
N$729: IC291.18(A:Y1)
N$730: IC291.16(A:Y2)
N$731: IC291.14(A:Y3)
N$732: IC291.12(A:Y4)
N$733: IC290.18(A:Y1)
N$734: IC290.16(A:Y2)
N$735: IC290.14(A:Y3)
N$736: IC290.12(A:Y4)
N$737: IC288.2(A:A1) IC291.2(A:A1) IC292.2(A:A1) IC301.2(1Q)
N$738: IC288.4(A:A2) IC291.4(A:A2) IC292.4(A:A2) IC301.5(2Q)
N$739: IC288.6(A:A3) IC291.6(A:A3) IC292.6(A:A3) IC301.6(3Q)
N$740: IC288.8(A:A4) IC291.8(A:A4) IC292.8(A:A4) IC301.9(4Q)
N$741: IC289.2(A:A1) IC290.2(A:A1) IC293.2(A:A1) IC301.12(5Q)
N$742: IC289.4(A:A2) IC290.4(A:A2) IC293.4(A:A2) IC301.15(6Q)
N$743: IC289.6(A:A3) IC290.6(A:A3) IC293.6(A:A3) IC301.16(7Q)
N$744: IC289.8(A:A4) IC290.8(A:A4) IC293.8(A:A4) IC301.19(8Q)
N$745: IC292.18(A:Y1)
N$746: IC292.16(A:Y2)
N$747: IC292.14(A:Y3)
N$748: IC292.12(A:Y4)
N$749: IC293.18(A:Y1)
N$750: IC293.16(A:Y2)
N$751: IC293.14(A:Y3)
N$752: IC293.12(A:Y4)
N$753: IC295.2(A:A1) IC296.2(1Q) IC298.2(A:A1) IC299.2(A:A1)
N$754: IC295.4(A:A2) IC296.5(2Q) IC298.4(A:A2) IC299.4(A:A2)
N$755: IC295.6(A:A3) IC296.6(3Q) IC298.6(A:A3) IC299.6(A:A3)
N$756: IC295.8(A:A4) IC296.9(4Q) IC298.8(A:A4) IC299.8(A:A4)
N$757: IC294.2(A:A1) IC296.12(5Q) IC297.2(A:A1) IC300.2(A:A1)
N$758: IC294.4(A:A2) IC296.15(6Q) IC297.4(A:A2) IC300.4(A:A2)
N$759: IC294.6(A:A3) IC296.16(7Q) IC297.6(A:A3) IC300.6(A:A3)
N$760: IC294.8(A:A4) IC296.19(8Q) IC297.8(A:A4) IC300.8(A:A4)
N$761: IC285.4(S1) IC302.2(A1)
N$762: IC285.1(S2) IC302.3(A2)
N$763: IC285.13(S3) IC302.4(A3)
N$764: IC285.10(S4) IC302.5(A4)
N$765: IC283.4(S1) IC302.6(A5)
N$766: IC283.1(S2) IC302.7(A6)
N$767: IC283.13(S3) IC302.8(A7)
N$768: IC283.10(S4) IC302.9(A8)
N$769: IC284.4(S1) IC303.2(A1)
N$770: IC284.1(S2) IC303.3(A2)
N$771: IC284.13(S3) IC303.4(A3)
N$772: IC284.10(S4) IC303.5(A4)
N$773: IC286.4(S1) IC303.6(A5)
N$774: IC286.1(S2) IC303.7(A6)
N$775: IC286.13(S3) IC303.8(A7)
N$776: IC286.10(S4) IC303.9(A8)
N$777: IC28.2(A1) IC287.4(S1)
N$778: IC28.3(A2) IC287.1(S2)
N$779: IC28.4(A3) IC287.13(S3)
N$780: IC28.5(A4) IC287.10(S4)
NOT_CONDITION: IC74.4(B:I0)
NOT_RST: IC75.1(CLR) IC76.1(CLR) IC77.1(CLR) IC78.1(CLR) IC79.1(CLR) IC134.1(CLR) IC135.1(CLR) IC136.1(CLR) IC137.1(CLR)
OF: IC122.5(A4) IC156.10(2C0) IC227.9(Q4) IC256.6(1C0)
OF_FROM_ALU: IC126.8(4D) IC156.12(2C2) IC256.5(1C1)
OF_IN_SRC_0: IC256.14(A)
OF_IN_SRC_1: IC256.2(B)
PANEL_MEM_IO: RN4.3
PANEL_RD: RN4.1
PANEL_WR: RN4.2
PC_H_0: IC277.3(1B)
PC_H_1: IC277.6(2B)
PC_H_2: IC277.10(3B)
PC_H_3: IC277.13(4B)
PC_H_4: IC278.3(1B)
PC_H_5: IC278.6(2B)
PC_H_6: IC278.10(3B)
PC_H_7: IC278.13(4B)
PC_L_0: IC268.3(1B)
PC_L_1: IC268.6(2B)
PC_L_2: IC268.10(3B)
PC_L_3: IC268.13(4B)
PC_L_4: IC272.3(1B)
PC_L_5: IC272.6(2B)
PC_L_6: IC272.10(3B)
PC_L_7: IC272.13(4B)
PCH_0: IC6.2(1Q) IC107.11(B:A1)
PCH_1: IC6.5(2Q) IC107.13(B:A2)
PCH_2: IC6.6(3Q) IC107.15(B:A3)
PCH_3: IC6.9(4Q) IC107.17(B:A4)
PCH_4: IC6.12(5Q) IC108.11(B:A1)
PCH_5: IC6.15(6Q) IC108.13(B:A2)
PCH_6: IC6.16(7Q) IC108.15(B:A3)
PCH_7: IC6.19(8Q) IC108.17(B:A4)
PCH_OUT: IC107.19(B:G) IC108.19(B:G)
PCH_WRT: IC6.1(G)
PCL_0: IC48.2(1Q) IC105.11(B:A1)
PCL_1: IC48.5(2Q) IC105.13(B:A2)
PCL_2: IC48.6(3Q) IC105.15(B:A3)
PCL_3: IC48.9(4Q) IC105.17(B:A4)
PCL_4: IC48.12(5Q) IC106.11(B:A1)
PCL_5: IC48.15(6Q) IC106.13(B:A2)
PCL_6: IC48.16(7Q) IC106.15(B:A3)
PCL_7: IC48.19(8Q) IC106.17(B:A4)
PCL_OUT: IC105.19(B:G) IC106.19(B:G)
PCL_WRT: IC48.1(G)
PF: IC70.15(D4) IC122.9(A8) IC208.6(1C0) IC227.12(Q5)
PF_FROM_ALU: IC59.2(A:O) IC208.5(1C1)
PF_IN_SRC_0: IC208.14(A)
PF_IN_SRC_1: IC208.2(B)
PROG_MODE: IC250.5(B:I1)
RD: IC60.2(Q1) IC69.11(B:A1)
REQ_ENCOD_0: IC222.1(A)
REQ_ENCOD_1: IC154.6(A5) IC222.2(B) IC226.7(A1)
REQ_ENCOD_2: IC154.5(A4) IC222.3(C) IC226.6(A2)
RST: IC54.3(B:I) IC128.15(CLR) IC139.15(CLR) IC144.15(CLR) IC248.15(CLR) IC249.15(CLR) R3.1 S2.2(P)
SF: IC122.4(A3) IC156.6(1C0) IC227.6(Q3) IC255.6(1C0)
SF_FROM_ALU: IC126.7(3D) IC156.4(1C2)
SF_IN_SRC_0: IC255.14(A)
SF_IN_SRC_1: IC255.2(B)
SF_XOR_OF: IC70.14(D5) IC72.6(B:O) IC81.4(B:I0)
SHR_MACHINE_H_OUT: IC104.1(G1) IC104.19(G2)
SHR_MACHINE_H_WRT: IC82.1(G)
SHR_MACHINE_IN_SRC: IC94.1(!A!/B) IC95.1(!A!/B) IC96.1(!A!/B) IC97.1(!A!/B)
SHR_MACHINE_L_OUT: IC103.1(G1) IC103.19(G2)
SHR_MACHINE_L_WRT: IC93.1(G)
SHR_MACHINE_TYPE: IC161.2(A:I1)
SI_H_OUT: IC253.1(G1) IC253.19(G2)
SI_H_WRT: IC202.1(G)
SI_L_OUT: IC252.1(G1) IC252.19(G2)
SI_L_WRT: IC251.1(G)
SPH_OUT: IC111.19(B:G) IC112.19(B:G)
SPH_WRT: IC4.1(G)
SPL_OUT: IC109.19(B:G) IC110.19(B:G)
SPL_WRT: IC5.1(G)
SS_H_0: IC275.4(1C2)
SS_H_1: IC275.12(2C2)
SS_H_2: IC276.4(1C2)
SS_H_3: IC276.12(2C2)
SS_H_4: IC273.4(1C2)
SS_H_5: IC273.12(2C2)
SS_H_6: IC274.4(1C2)
SS_H_7: IC274.12(2C2)
SS_H_OUT: IC260.1(G1) IC260.19(G2)
SS_H_WRT: IC217.1(G)
SS_L_0: IC282.4(1C2)
SS_L_1: IC282.12(2C2)
SS_L_2: IC279.4(1C2)
SS_L_3: IC279.12(2C2)
SS_L_4: IC280.4(1C2)
SS_L_5: IC280.12(2C2)
SS_L_6: IC281.4(1C2)
SS_L_7: IC281.12(2C2)
SS_L_OUT: IC259.1(G1) IC259.19(G2)
SS_L_WRT: IC246.1(G)
STOP_CLK: IC44.2(A:D) IC44.5(A:Q) IC147.4(B:I0) R9.1 S4.2(P)
TDR0_H_WRT: IC239.1(G)
TDR0_H_X_OUT: IC237.1(A:G) IC238.1(A:G)
TDR0_L_WRT: IC240.1(G)
TDR0_L_X_OUT: IC235.8(A:A4)
TDR0H_WRT: IC17.1(G)
TDR0H_Y_OUT: IC213.1(A:G) IC214.1(A:G)
TDR0L_OUT3: IC229.1(A:G)
TDR0L_OUT4: IC235.1(A:G)
TDR0L_WRT: IC16.1(G)
TDR0L_Y_OUT: IC211.1(A:G) IC212.1(A:G)
TDR1_H_WRT: IC233.1(G)
TDR1_H_X_OUT: IC231.1(A:G) IC232.1(A:G)
TDR1_L_WRT: IC234.1(G)
TDR1_L_X_OUT: IC229.8(A:A4)
TDR1H_WRT: IC88.1(G)
TDR1H_Y_OUT: IC91.1(A:G) IC92.1(A:G)
TDR1L_WRT: IC86.1(G)
TDR1L_Y_OUT: IC89.1(A:G) IC90.1(A:G)
TRAP: IC45.2(A:I1)
TRAP_REQ: IC8.3(A:CLK) IC148.1(A:I0) R5.2
TRISTATE: IC28.1(G1) IC28.19(G2) IC69.19(B:G) IC250.6(B:O) IC302.1(G1) IC302.19(G2) IC303.1(G1) IC303.19(G2)
TYP_0: IC43.3(B:I) IC67.4(B:I0) IC85.1(A:I0)
TYP_1: IC39.2(A:I1) IC42.1(A:I0) IC84.3(B:I)
U_AD0: IC32.2(Q1) U$6.10(A0) U$7.10(A0) U$8.10(A0) U$9.10(A0)
U_AD1: IC32.5(Q2) U$6.9(A1) U$7.9(A1) U$8.9(A1) U$9.9(A1)
U_AD2: IC32.6(Q3) U$6.8(A2) U$7.8(A2) U$8.8(A2) U$9.8(A2)
U_AD3: IC32.9(Q4) U$6.7(A3) U$7.7(A3) U$8.7(A3) U$9.7(A3)
U_AD4: IC32.12(Q5) U$6.6(A4) U$7.6(A4) U$8.6(A4) U$9.6(A4)
U_AD5: IC32.15(Q6) U$6.5(A5) U$7.5(A5) U$8.5(A5) U$9.5(A5)
U_AD6: IC32.16(Q7) U$6.4(A6) U$7.4(A6) U$8.4(A6) U$9.4(A6)
U_AD7: IC32.19(Q8) U$6.3(A7) U$7.3(A7) U$8.3(A7) U$9.3(A7)
U_AD8: IC33.2(Q1) U$6.25(A8) U$7.25(A8) U$8.25(A8) U$9.25(A8)
U_AD9: IC33.5(Q2) U$6.24(A9) U$7.24(A9) U$8.24(A9) U$9.24(A9)
U_AD10: IC33.6(Q3) U$6.21(A10) U$7.21(A10) U$8.21(A10) U$9.21(A10)
U_AD11: IC33.9(Q4) U$6.23(A11) U$7.23(A11) U$8.23(A11) U$9.23(A11)
U_AD12: IC33.12(Q5) U$6.2(A12) U$7.2(A12) U$8.2(A12) U$9.2(A12)
U_AD13: IC33.15(Q6) U$6.26(A13) U$7.26(A13) U$8.26(A13) U$9.26(A13)
U_AD14: IC33.16(Q7)
U_AD15: IC33.19(Q8)
U_AD_BUFF0: U$1.10(A0)
U_AD_BUFF1: U$1.9(A1)
U_AD_BUFF2: U$1.8(A2)
U_AD_BUFF3: U$1.7(A3)
U_AD_BUFF4: U$1.6(A4)
U_AD_BUFF5: U$1.5(A5)
U_AD_BUFF6: U$1.4(A6)
U_AD_BUFF7: U$1.3(A7)
U_AD_BUFF8: U$1.25(A8)
U_AD_BUFF9: U$1.24(A9)
U_AD_BUFF10: U$1.21(A10)
U_AD_BUFF11: U$1.23(A11)
U_AD_BUFF12: U$1.2(A12)
U_AD_BUFF13: U$1.26(A13)
U_ADDER_0: IC50.4(S1) IC186.4(D0)
U_ADDER_1: IC160.4(D0)
U_ADDER_2: IC159.4(D0)
U_ADDER_3: IC142.4(D0)
U_ADDER_4: IC129.4(D0)
U_ADDER_5: IC73.4(D0)
U_ADDER_6: IC34.4(D0)
U_ADDER_7: IC35.4(D0)
U_ADDER_8: IC36.4(D0)
U_ADDER_9: IC37.4(D0)
U_ADDER_10: IC38.4(D0)
U_ADDER_11: IC40.4(D0)
U_ADDER_12: IC41.4(D0)
U_ADDER_13: IC53.1(S2) IC71.4(D0)
U_ADDER_14: IC20.4(D0)
U_ADDER_15: IC172.4(D0)
U_ADDR_MUX_1: IC42.3(A:O)
U_CF: IC126.5(2Q) IC155.11(2C1) IC167.3(1B)
U_DMA_0: IC186.14(D5)
U_DMA_1: IC160.14(D5)
U_DMA_2: IC159.14(D5)
U_DMA_3: IC142.14(D5)
U_DMA_4: IC129.14(D5)
U_DMA_5: IC73.14(D5)
U_DMA_6: IC34.14(D5)
U_DMA_7: IC35.14(D5)
U_DMA_8: IC36.14(D5)
U_DMA_9: IC37.14(D5)
U_DMA_10: IC38.14(D5)
U_DMA_11: IC40.14(D5)
U_DMA_12: IC41.14(D5)
U_DMA_13: IC71.14(D5)
U_DMA_14: IC20.14(D5)
U_DMA_15: IC172.14(D5)
U_FETCH_0: IC186.2(D2)
U_FETCH_1: IC160.2(D2)
U_FETCH_2: IC159.2(D2)
U_FETCH_3: IC142.2(D2)
U_FETCH_4: IC129.2(D2)
U_FETCH_5: IC73.2(D2)
U_FETCH_6: IC34.2(D2)
U_FETCH_7: IC35.2(D2)
U_FETCH_8: IC36.2(D2)
U_FETCH_9: IC37.2(D2)
U_FETCH_10: IC38.2(D2)
U_FETCH_11: IC40.2(D2)
U_FETCH_12: IC41.2(D2)
U_FETCH_13: IC71.2(D2)
U_FETCH_14: IC20.2(D2)
U_FETCH_15: IC172.2(D2)
U_FLAGS_REG_WRT: IC126.1(G)
U_INTERRUPT_0: IC186.1(D3)
U_INTERRUPT_1: IC160.1(D3)
U_INTERRUPT_2: IC159.1(D3)
U_INTERRUPT_3: IC142.1(D3)
U_INTERRUPT_4: IC129.1(D3)
U_INTERRUPT_5: IC73.1(D3)
U_INTERRUPT_6: IC34.1(D3)
U_INTERRUPT_7: IC35.1(D3)
U_INTERRUPT_8: IC36.1(D3)
U_INTERRUPT_9: IC37.1(D3)
U_INTERRUPT_10: IC38.1(D3)
U_INTERRUPT_11: IC40.1(D3)
U_INTERRUPT_12: IC41.1(D3)
U_INTERRUPT_13: IC71.1(D3)
U_INTERRUPT_14: IC20.1(D3)
U_INTERRUPT_15: IC172.1(D3)
U_OF: IC126.9(4Q) IC156.11(2C1)
U_OFFSET0: IC49.3(1B)
U_OFFSET1: IC49.6(2B)
U_OFFSET2: IC49.10(3B)
U_OFFSET3: IC49.13(4B)
U_OFFSET4: IC55.3(1B)
U_OFFSET5: IC55.6(2B)
U_OFFSET6: IC55.10(3B)
U_SF: IC126.6(3Q) IC156.5(1C1)
U_TRAP_0: IC186.15(D4)
U_TRAP_1: IC160.15(D4)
